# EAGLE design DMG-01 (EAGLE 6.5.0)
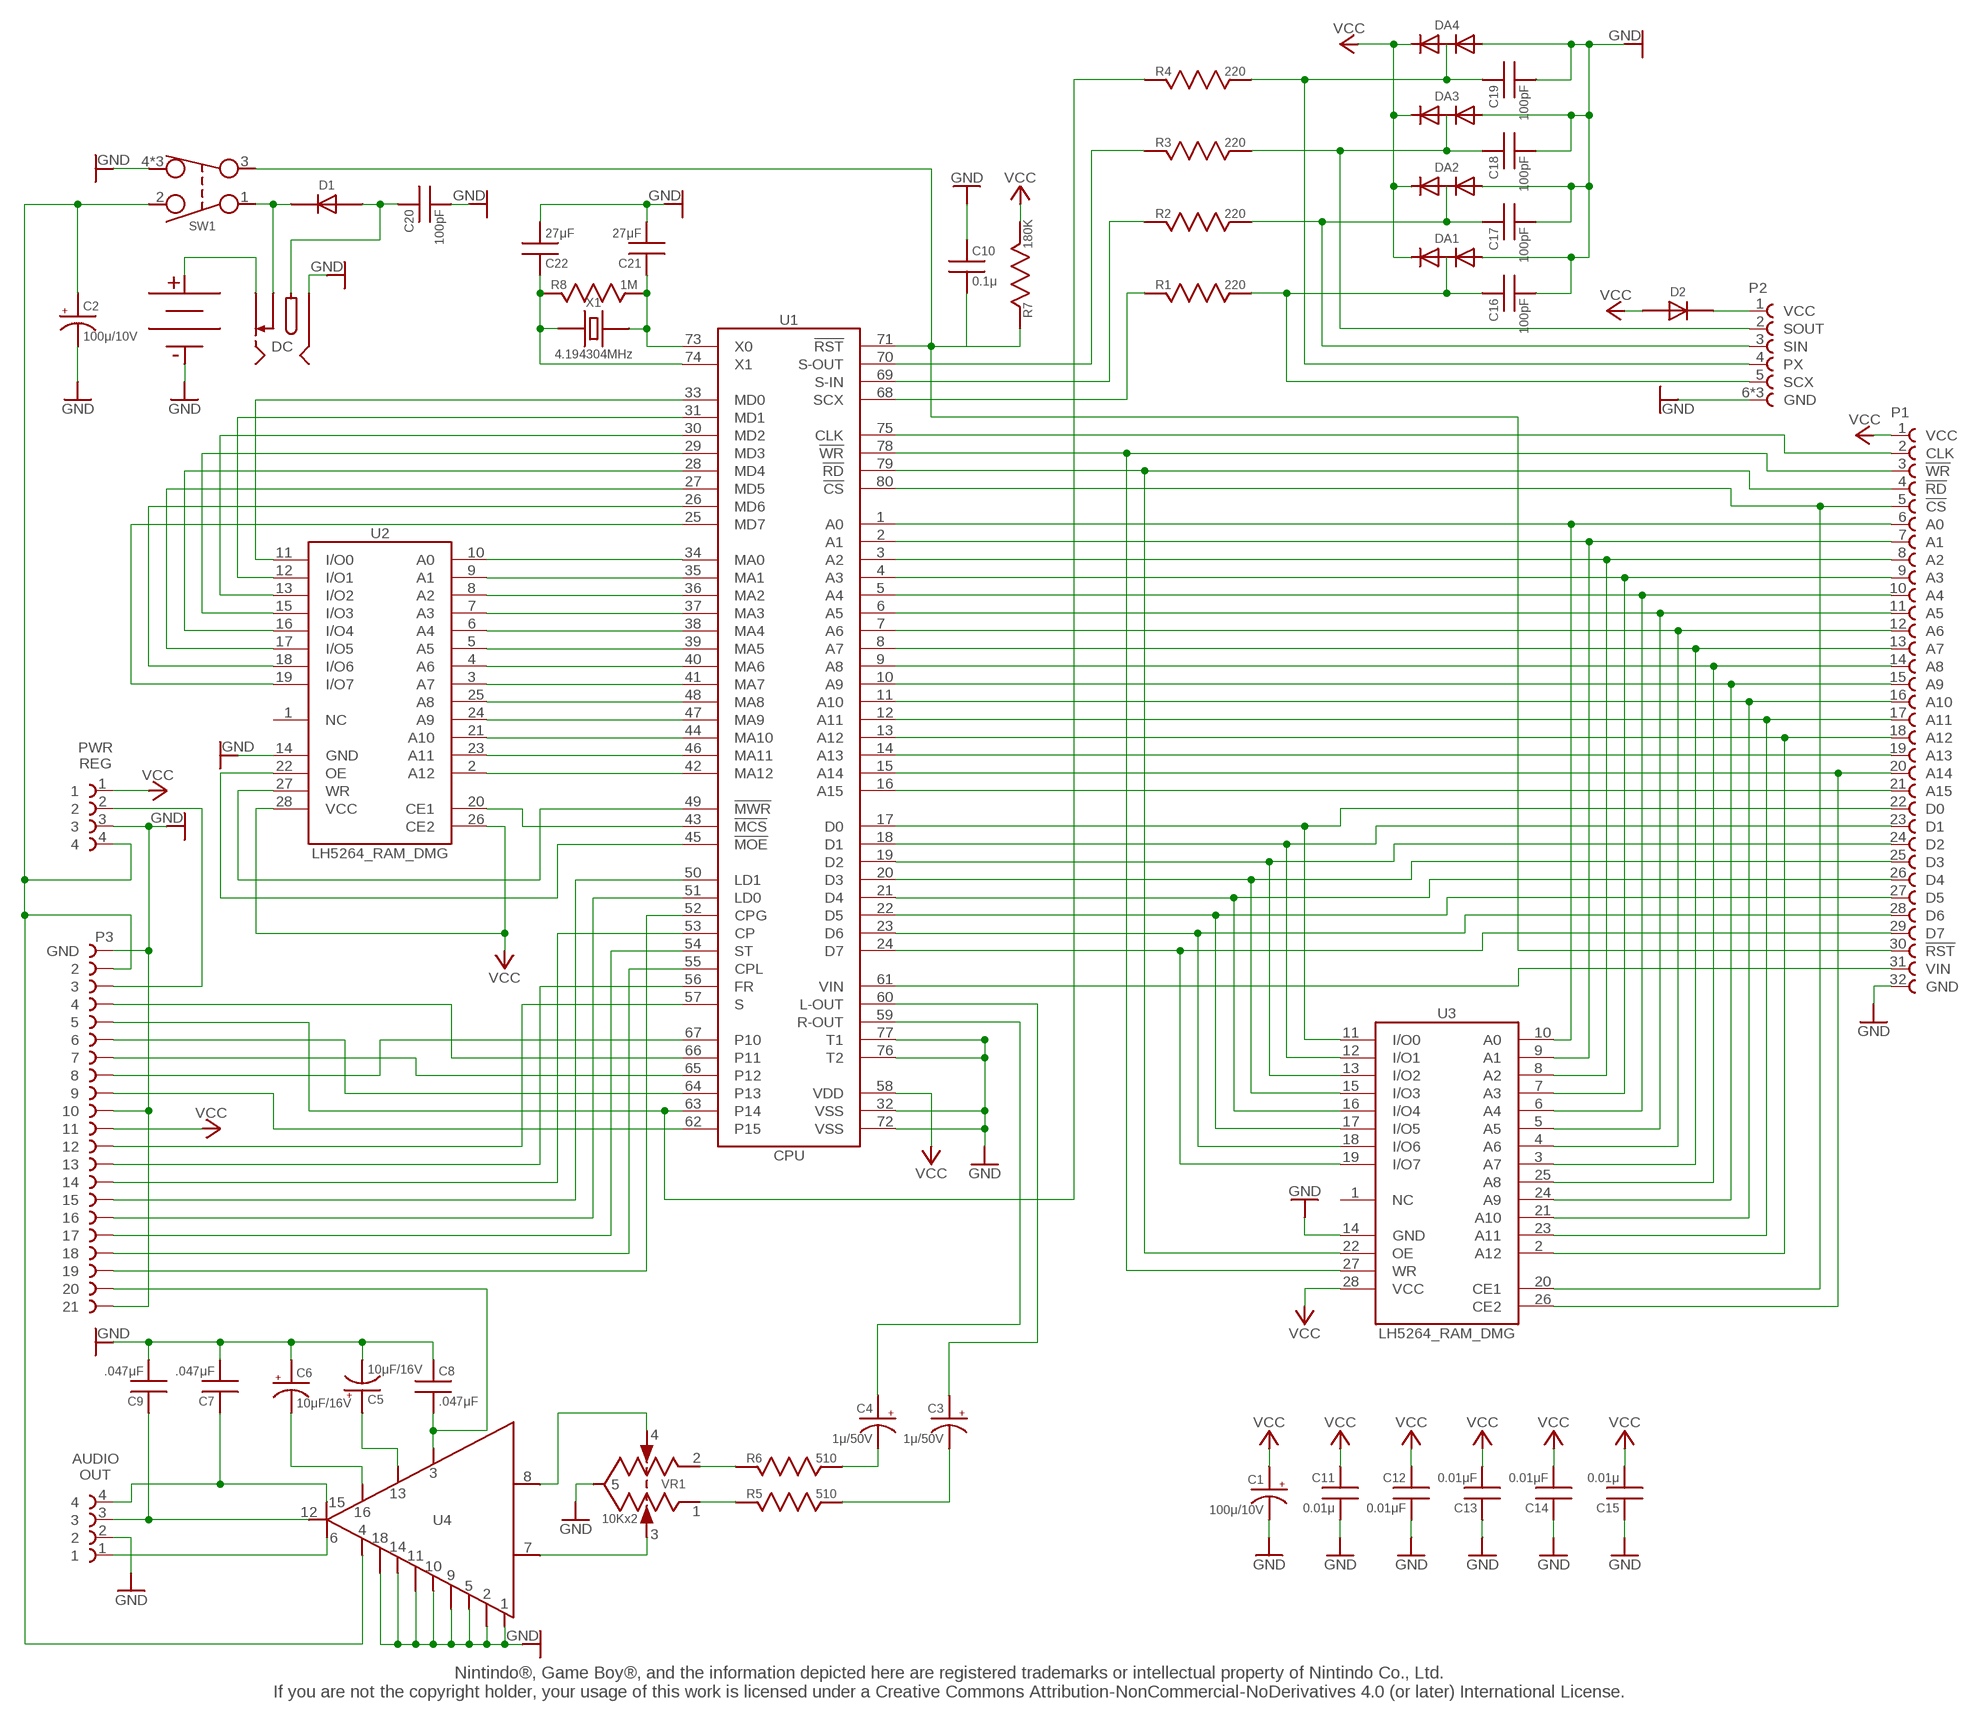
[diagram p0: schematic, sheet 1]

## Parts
C1  100μ/10V  CAPACITOR_ELECTROLYTIC_200MIL  [CAP-200E]
C2  100μ/10V  CAPACITOR_ELECTROLYTIC_200MIL  [CAP-200E]
C3  1μ/50V  CAPACITOR_ELECTROLYTIC_200MIL  [CAP-200E]
C4  1μ/50V  CAPACITOR_ELECTROLYTIC_200MIL  [CAP-200E]
C5  10μF/16V  CAPACITOR_ELECTROLYTIC_200MIL  [CAP-200E]
C6  10μF/16V  CAPACITOR_ELECTROLYTIC_200MIL  [CAP-200E]
C7  .047μF  CAPACITOR_200MIL  [CAP-200]
C8  .047μF  CAPACITOR_200MIL  [CAP-200]
C9  .047μF  CAPACITOR_200MIL  [CAP-200]
C10  0.1μ  CAPACITOR_200MIL  [CAP-200]
C11  0.01μ  CAPACITOR_200MIL  [CAP-200]
C12  0.01μF  CAPACITOR_200MIL  [CAP-200]
C13  0.01μF  CAPACITOR_200MIL  [CAP-200]
C14  0.01μF  CAPACITOR_200MIL  [CAP-200]
C15  0.01μ  CAPACITOR_200MIL  [CAP-200]
C16  100pF  CAPACITOR_100MIL  [CAP-100]
C17  100pF  CAPACITOR_100MIL  [CAP-100]
C18  100pF  CAPACITOR_100MIL  [CAP-100]
C19  100pF  CAPACITOR_100MIL  [CAP-100]
C20  100pF  CAPACITOR_100MIL  [CAP-100]
C21  27μF  CAPACITOR_100MIL  [CAP-100]
C22  27μF  CAPACITOR_100MIL  [CAP-100]
D1  DIODE_300MIL  [DIODE-300]
D2  DIODE_300MIL  [DIODE-300]
DA1  DIODE_ARRAY_DMG  [DMG_DIODE_ARRAY]
DA2  DIODE_ARRAY_DMG  [DMG_DIODE_ARRAY]
DA3  DIODE_ARRAY_DMG  [DMG_DIODE_ARRAY]
DA4  DIODE_ARRAY_DMG  [DMG_DIODE_ARRAY]
DC  PWR_JACK_DMG  [DMG_PWR_JACK]
P1  DMG_SOCKET  [DMG_SOCKET]
P2  DMG_LINK_PORT  [DMG_LINK_PORT]
P3  DMG_SOCKET_SCREEN  [DMG_SOCKET_SCREEN]
R1  220  RESISTOR600MIL  [RES-300]
R2  220  RESISTOR600MIL  [RES-300]
R3  220  RESISTOR600MIL  [RES-300]
R4  220  RESISTOR600MIL  [RES-300]
R5  510  RESISTOR600MIL  [RES-300]
R6  510  RESISTOR600MIL  [RES-300]
R7  180K  RESISTOR600MIL  [RES-300]
R8  1M  RESISTOR600MIL  [RES-300]
SW1  SWITCH_DMG  [DMG_SWITCH]
U1  CPU  LR35902_CPU_DMG  [LR35902_CPU_DMG]
U2  LH5264_RAM_DMG  [LH5264_RAM_DMG]
U3  LH5264_RAM_DMG  [LH5264_RAM_DMG]
U4  AMP_DMG  [AMP_DMG]
U$3  DMG_OUTBOARD  [DMG_OUTBOARD]
U$6  BAT+_DMG  [DMG_BAT+]
U$7  DMG_OUTBOARD  [DMG_OUTBOARD]
U$8  BAT-_DMG  [DMG_BAT-]
VR1  10Kx2  POT_DMG_DMG  [DMG_POT]
X1  4.194304MHz  CLOCK_DMG  [CLOCK_DMG]

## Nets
BAT: DC.4 U$6.POS(BAT+)
GND: C1.2(-) C2.2(-) C5.2(-) C6.1(+) C7.2 C8.1 C9.2 C10.1 C11.2 C12.2 C13.1 C14.1 C15.1 C16.2 C17.2 C18.2 C19.2 C20.2 C21.2 C22.2 DA1.1 DA2.1 DA3.1 DA4.1 DC.1 P1.32(GND) P2.6(GND) P2.MT1(GND) P2.MT2(GND) P3.1(GND) P3.10 P3.21 SW1.4 SW1.MT1 SW1.MT2 U1.32(VSS) U1.72(VSS) U1.76(T2) U1.77(T1) U2.14(GND) U3.14(GND) U4.1 U4.2 U4.5 U4.9 U4.10 U4.11 U4.14 U4.18 U$3.2 U$7.3 U$8.NEG(BAT-) VR1.5 VR1.MT1 VR1.MT2 ; supply symbol labelled GND_SIDE, GND_END
L-OUT: C3.1(+) U1.60(L-OUT)
L-STEP1: C3.2(-) R5.2
L-STEP2: R5.1 VR1.1
L-STEP3: U4.7 VR1.3
LEFT: C7.1 U4.15 U$3.4
N$1: P1.31(VIN) U1.61(VIN)
N$2: P3.3 U$7.2
N$3: D2.2 P2.1(VCC)
N$4: P1.29(D7) U1.24(D7) U3.19(I/O7)
N$5: P1.28(D6) U1.23(D6) U3.18(I/O6)
N$6: P1.27(D5) U1.22(D5) U3.17(I/O5)
N$7: P1.26(D4) U1.21(D4) U3.16(I/O4)
N$8: P1.25(D3) U1.20(D3) U3.15(I/O3)
N$9: P1.24(D2) U1.19(D2) U3.13(I/O2)
N$10: P1.23(D1) U1.18(D1) U3.12(I/O1)
N$11: P1.22(D0) U1.17(D0) U3.11(I/O0)
N$12: P1.21(A15) U1.16(A15)
N$13: P1.20(A14) U1.15(A14) U3.26(CE2)
N$14: P1.19(A13) U1.14(A13)
N$15: P1.18(A12) U1.13(A12) U3.2(A12)
N$16: P1.17(A11) U1.12(A11) U3.23(A11)
N$17: P1.16(A10) U1.11(A10) U3.21(A10)
N$18: P1.15(A9) U1.10(A9) U3.24(A9)
N$19: P1.14(A8) U1.9(A8) U3.25(A8)
N$20: P1.13(A7) U1.8(A7) U3.3(A7)
N$21: P1.12(A6) U1.7(A6) U3.4(A6)
N$22: P1.11(A5) U1.6(A5) U3.5(A5)
N$23: P1.10(A4) U1.5(A4) U3.6(A4)
N$24: P1.9(A3) U1.4(A3) U3.7(A3)
N$25: P1.8(A2) U1.3(A2) U3.8(A2)
N$26: P1.7(A1) U1.2(A1) U3.9(A1)
N$27: P1.6(A0) U1.1(A0) U3.10(A0)
N$28: P1.5(!CS) U1.80(!CS) U3.20(CE1)
N$29: P1.4(!RD) U1.79(!RD) U3.22(OE)
N$30: P1.2(CLK) U1.75(CLK)
N$31: U1.33(MD0) U2.11(I/O0)
N$32: U1.31(MD1) U2.12(I/O1)
N$33: U1.30(MD2) U2.13(I/O2)
N$34: U1.29(MD3) U2.15(I/O3)
N$35: U1.28(MD4) U2.16(I/O4)
N$36: U1.27(MD5) U2.17(I/O5)
N$37: U1.26(MD6) U2.18(I/O6)
N$38: U1.25(MD7) U2.19(I/O7)
N$39: U1.45(!MOE) U2.22(OE)
N$40: U1.49(!MWR) U2.27(WR)
N$41: U1.43(!MCS) U2.20(CE1)
N$42: U1.42(MA12) U2.2(A12)
N$43: U1.46(MA11) U2.23(A11)
N$44: U1.44(MA10) U2.21(A10)
N$45: U1.47(MA9) U2.24(A9)
N$46: U1.48(MA8) U2.25(A8)
N$47: U1.41(MA7) U2.3(A7)
N$48: U1.40(MA6) U2.4(A6)
N$49: U1.39(MA5) U2.5(A5)
N$50: U1.38(MA4) U2.6(A4)
N$51: U1.37(MA3) U2.7(A3)
N$52: U1.36(MA2) U2.8(A2)
N$53: U1.35(MA1) U2.9(A1)
N$54: U1.34(MA0) U2.10(A0)
N$55: C21.1 R8.2 U1.73(X0) X1.2
N$56: C22.1 R8.1 U1.74(X1) X1.1
N$57: P1.3(!WR) U1.78(!WR) U3.27(WR)
N$58: R3.1 U1.70(S-OUT)
N$59: R2.1 U1.69(S-IN)
N$60: P3.5 R4.1 U1.63(P14)
N$61: R1.1 U1.68(SCX)
N$62: C16.1 DA1.2 P2.5(SCX) R1.2
N$63: C17.1 DA2.2 P2.3(SIN) R2.2
N$64: C18.1 DA3.2 P2.2(SOUT) R3.2
N$65: C19.1 DA4.2 P2.4(PX) R4.2
N$77: U4.6 U$3.1
N$78: C6.2(-) U4.16
N$79: C8.2 P3.20 U4.3
N$80: P3.4 U1.66(P11)
N$81: P3.6 U1.64(P13)
N$82: P3.7 U1.65(P12)
N$83: P3.8 U1.67(P10)
N$84: P3.9 U1.62(P15)
N$85: P3.12 U1.57(S)
N$86: P3.13 U1.56(FR)
N$87: P3.14 U1.53(CP)
N$88: P3.15 U1.50(LD1)
N$89: P3.16 U1.51(LD0)
N$90: P3.17 U1.54(ST)
N$91: P3.18 U1.55(CPL)
N$92: P3.19 U1.52(CPG)
N$102: C5.1(+) U4.13
N$106: C20.1 D1.1 DC.2
PWR: C2.1(+) D1.2 DC.3 P3.2 SW1.1 SW1.2 U4.4 U$7.4
R-OUT: C4.1(+) U1.59(R-OUT)
R-STEP1: C4.2(-) R6.2
R-STEP2: R6.1 VR1.2
R-STEP3: U4.8 VR1.4
RIGHT: C9.1 U4.12 U$3.3
RST: C10.2 P1.30(!RST) R7.1 SW1.3 U1.71(!RST)
VCC: C1.1(+) C11.1 C12.1 C13.2 C14.2 C15.2 D2.1 DA1.3 DA2.3 DA3.3 DA4.3 P1.1(VCC) P3.11 R7.2 U1.58(VDD) U2.26(CE2) U2.28(VCC) U3.28(VCC) U$7.1 ; supply symbol labelled VCC_END
Unconnected: U2.1(NC) U3.1(NC)

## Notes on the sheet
- PWR
  REG
- AUDIO
  OUT
- Nintindo®, Game Boy®, and the information depicted here are registered trademarks or intellectual property of Nintindo Co., Ltd.
  If you are not the copyright holder, your usage of this work is licensed under a Creative Commons Attribution-NonCommercial-NoDerivatives 4.0 (or later) International License.

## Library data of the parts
C1-C6 = !custom:CAPACITOR_ELECTROLYTIC: DMG Electrolytic Capacitor
C7-C22 = !custom:CAPACITOR: Capacitor.
D1 D2 = !custom:DIODE: Diodes.
DA1-DA4 = !custom:DIODE_ARRAY_DMG: Used in DMG-01 for link-port sanitization.
DC = !custom:PWR_JACK_DMG: DC Power Jack used in DMG.
P1 = !custom:DMG_SOCKET: DMG Socket 32 Pin Cartridge Socket used in DMG-01
P2 = !custom:DMG_LINK_PORT: DMG Link port; used to communicate with other Gameboys.
P3 = !custom:DMG_SOCKET_SCREEN: DMG Flex Cable Connecter This part does not have any spec that can be found. Part was measured with a caliper with a resolution of .5mil. Pad spacing is at 50mil.
R1-R8 = !custom:RESISTOR: Resistor.
SW1 = !custom:SWITCH_DMG: Power switch used in DMG.
U1 = !custom:LR35902_CPU: Sharp LR35902 CPU Z80/8080 Hybrid used in the DMG-01 The origional spec cannot be found, so assumptions are made. This thin quad flat pack (TQFP) uses a common spacing of 0.8mm between the pins. When compaired to a scaled photo, the solder pads match very closely.
U2 U3 = !custom:LH5264_RAM: LH5264 RAM Memory used in DMG-01 Original spec sheet cannot be found. This part is based off a currently used SHARP 28SOP footprint (SOP025-P-0450). When compared to scaled photo of DMG pads, this footprint's center of tolerance matches perfectly. Pads extended to 2mm.
U4 = !custom:AMP_DMG: Gameboy Audio Amp. There is no information on this that can be found. All measurements were taken with a caliper with a resolution of 0.01mm/.5mil. Measurements were attempted in both mm and mil. The closest round number was chosen for every dimension, then re-measured for accuracy.
U$3 U$7 = !custom:DMG_OUTBOARD: Solder holes for connections to auxiliary boards.
U$6 = !custom:BAT+_DMG: Positive battery contact for DMG.
U$8 = !custom:BAT-_DMG: Negative battery contact for DMG.
VR1 = !custom:POT_DMG: Volume/Contrast Potentiomentor used on DMG-01. Based off a common thumb-wheel potentiometer that matches board.
X1 = !custom:CLOCK: Crystal Oscillator.

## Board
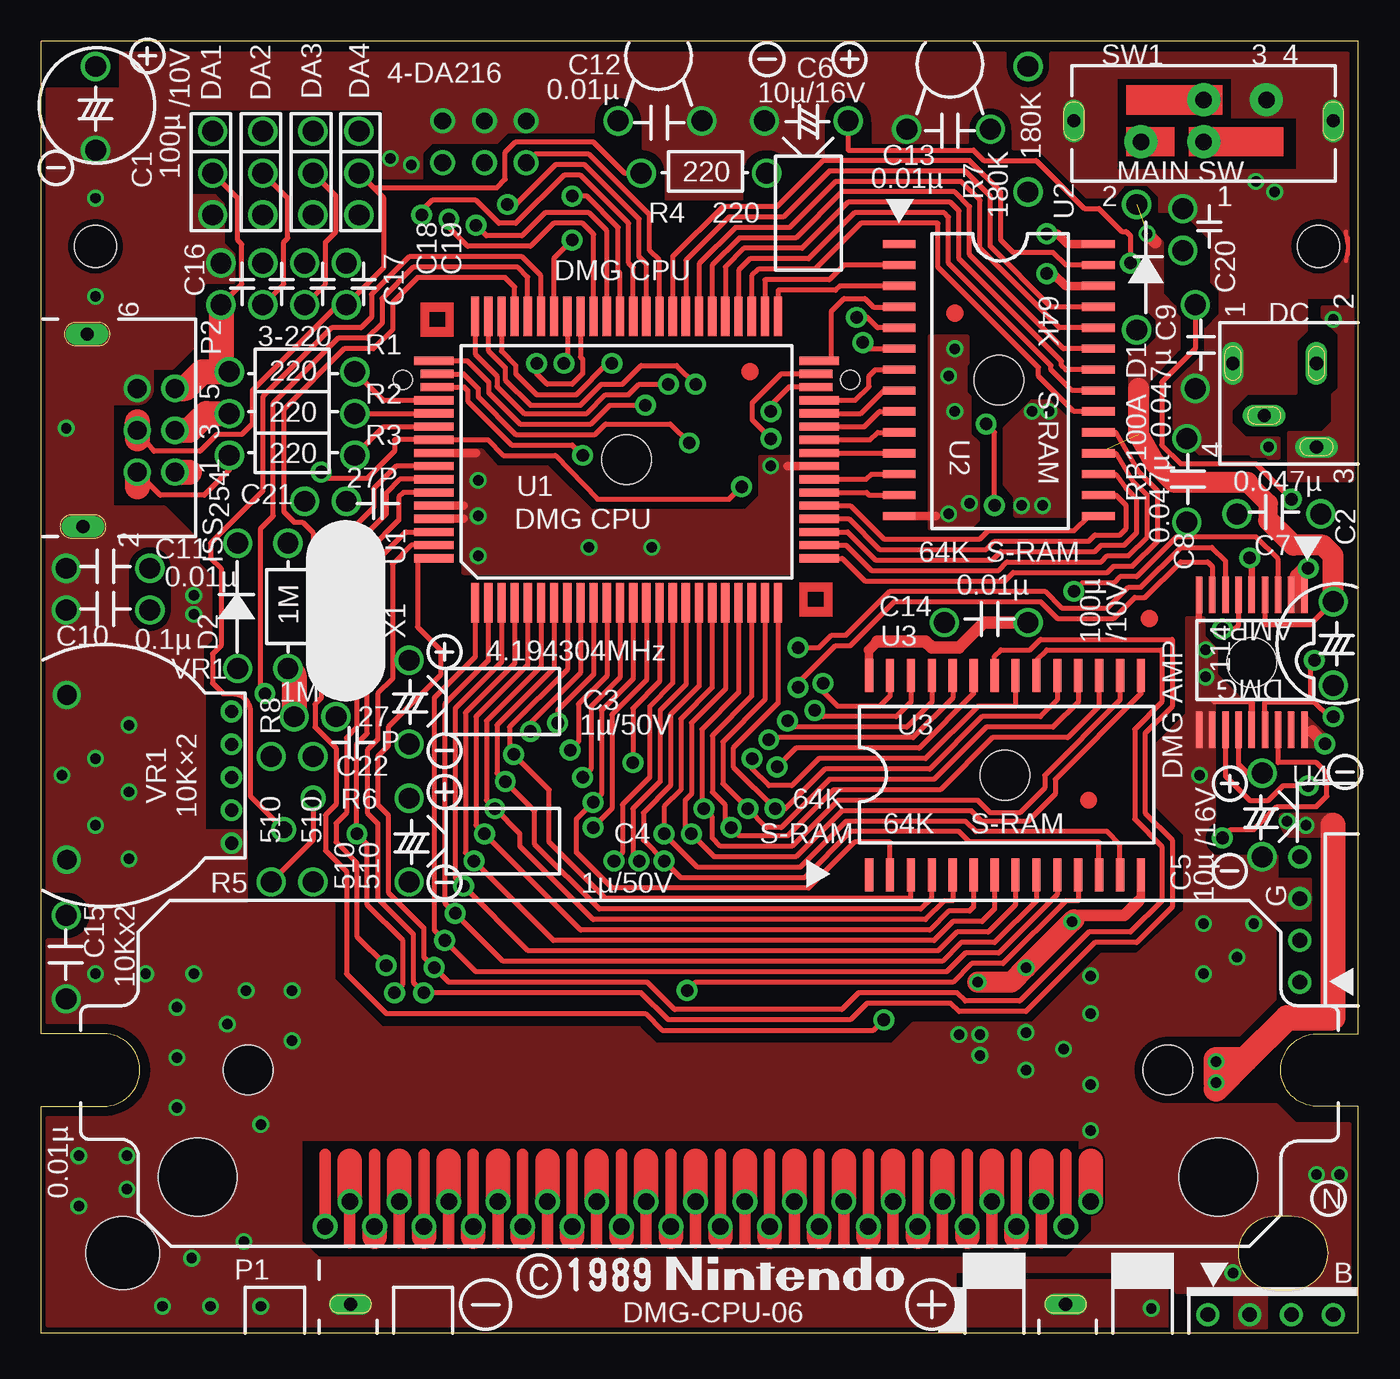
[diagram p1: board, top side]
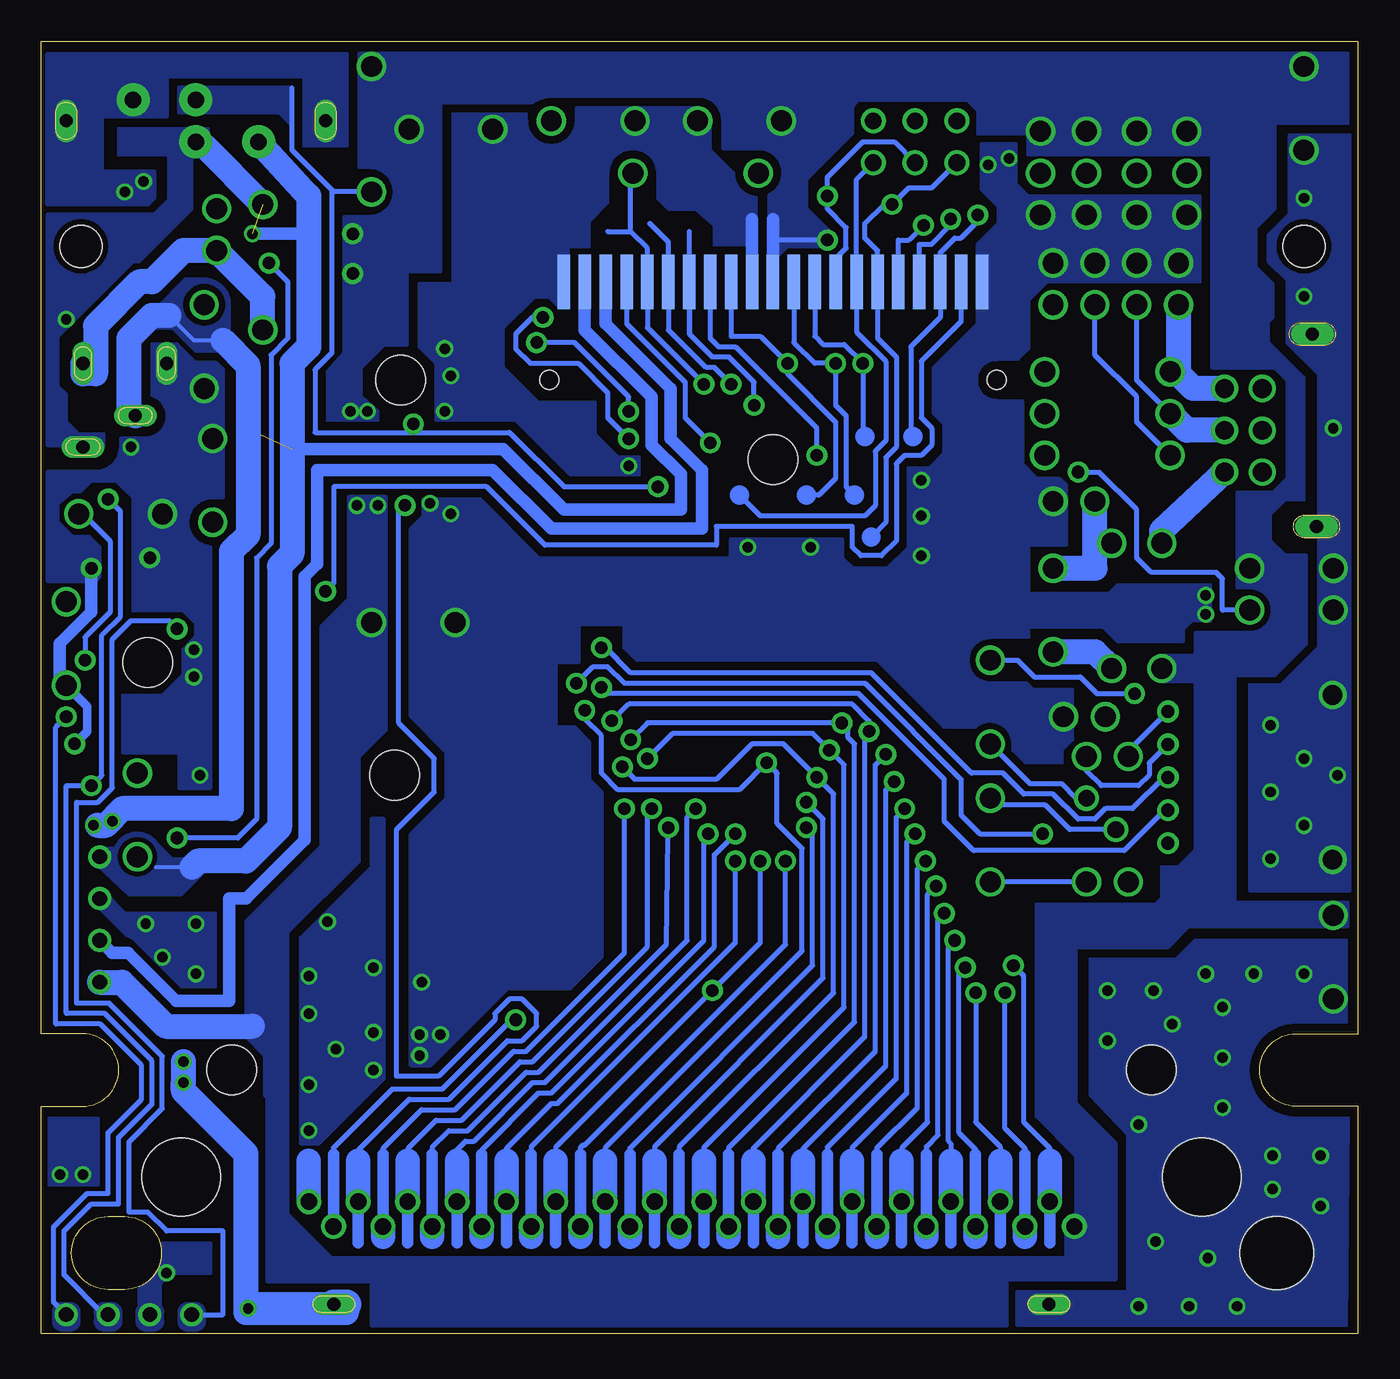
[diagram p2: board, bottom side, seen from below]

Size 80 x 78.5 mm. Coordinates in mm from the lower left corner, seen from the top.
Outline: 80,0 80,13.8 77.5,13.8 arc-180 77.5,18.2 80,18.2 80,78.5 0,78.5 0,18.2 3.8,18.2 arc-180 3.8,13.8 0,13.8 0,0 80,0
Copper layers (1*16): Top 0.035mm / dielectric 1.5mm / Bottom 0.035mm
Design rules "default *": minimum track width 10mil, minimum drill 24mil, track to track 5mil, track to pad 5mil, pad to pad 5mil, via to via 5mil, smd to smd 5mil, copper to edge 0mil, drill to drill 8mil, minimum pad ring 10mil, minimum via ring 1mil, stop-mask expansion 0mil, vias tented up to drill 0mil, thermal gap 0mil
Holes 2.54 mm at 3.3,66.04 77.6,66.04
Holes 4.45 mm at 4.95,4.89
Milling: 4 lines

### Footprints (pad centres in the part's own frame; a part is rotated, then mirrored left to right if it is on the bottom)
CAP-200E = drill 1.27: 1 -2.54,0; 2 2.54,0
CAP-200 = drill 1.27: 1 -2.54,0; 2 2.54,0
CAP-100 = drill 1.27: 1 -1.27,0; 2 1.27,0
DIODE-300 = drill 1.27: 1 3.81,0; 2 -3.81,0
DMG_DIODE_ARRAY = drill 1.27: 1 -2.54,0; 2 0,0; 3 2.54,0
DMG_PWR_JACK = drill 0.8 long: 1 -1.905,-2.54; 2 -1.905,2.54; 3 3.175,2.54; 4 1.27,-0.635
DMG_SOCKET = drill 1 pad 1.5: 1 -23.25,-9.5; 2 -21.75,-8; 3 -20.25,-9.5; 4 -18.75,-8; 5 -17.25,-9.5; 6 -15.75,-8; 7 -14.25,-9.5; 8 -12.75,-8; 9 -11.25,-9.5; 10 -9.75,-8; 11 -8.25,-9.5; 12 -6.75,-8; 13 -5.25,-9.5; 14 -3.75,-8; 15 -2.25,-9.5; 16 -0.75,-8; 17 0.75,-9.5; 18 2.25,-8; 19 3.75,-9.5; 20 5.25,-8; 21 6.75,-9.5; 22 8.25,-8; 23 9.75,-9.5; 24 11.25,-8; 25 12.75,-9.5; 26 14.25,-8; 27 15.75,-9.5; 28 17.25,-8; 29 18.75,-9.5; 30 20.25,-8; 31 21.75,-9.5; 32 23.25,-8 | hole 3: -27.925,0; 27.925,0 | hole 4.75: -31,-6.5; 31,-6.5
DMG_LINK_PORT = drill 1.143 pad 1.422: 1 7.366,-2.54; 2 5.08,-2.54; 3 7.366,0; 4 5.08,0; 5 7.366,2.54; 6 5.08,2.54 | drill 0.8 long: MT1 1.778,-5.842; MT2 2.032,5.842
DMG_SOCKET_SCREEN = smd 0.762 x 3.302: 1 -12.7,5.969; 2 -11.43,5.969; 3 -10.16,5.969; 4 -8.89,5.969; 5 -7.62,5.969; 6 -6.35,5.969; 7 -5.08,5.969; 8 -3.81,5.969; 9 -2.54,5.969; 10 -1.27,5.969; 11 0,5.969; 12 1.27,5.969; 13 2.54,5.969; 14 3.81,5.969; 15 5.08,5.969; 16 6.35,5.969; 17 7.62,5.969; 18 8.89,5.969; 19 10.16,5.969; 20 11.43,5.969; 21 12.7,5.969 | hole 1.143: -13.589,0; 13.589,0
RES-300 = drill 1.27: 1 -3.81,0; 2 3.81,0
DMG_SWITCH = drill 1 pad 2: 1 0,-1.27; 2 -3.81,-1.27; 3 0,1.27; 4 3.81,1.27 | drill 0.8 long: MT1 -7.874,0; MT2 7.874,0
LR35902_CPU_DMG = smd 0.5 x 2.4: 1 -9.2,-8.7; 2 -8.4,-8.7; 3 -7.6,-8.7; 4 -6.8,-8.7; 5 -6,-8.7; 6 -5.2,-8.7; 7 -4.4,-8.7; 8 -3.6,-8.7; 9 -2.8,-8.7; 10 -2,-8.7; 11 -1.2,-8.7; 12 -0.4,-8.7; 13 0.4,-8.7; 14 1.2,-8.7; 15 2,-8.7; 16 2.8,-8.7; 17 3.6,-8.7; 18 4.4,-8.7; 19 5.2,-8.7; 20 6,-8.7; 21 6.8,-8.7; 22 7.6,-8.7; 23 8.4,-8.7; 24 9.2,-8.7; 41 9.2,8.7; 42 8.4,8.7; 43 7.6,8.7; 44 6.8,8.7; 45 6,8.7; 46 5.2,8.7; 47 4.4,8.7; 48 3.6,8.7; 49 2.8,8.7; 50 2,8.7; 51 1.2,8.7; 52 0.4,8.7; 53 -0.4,8.7; 54 -1.2,8.7; 55 -2,8.7; 56 -2.8,8.7; 57 -3.6,8.7; 58 -4.4,8.7; 59 -5.2,8.7; 60 -6,8.7; 61 -6.8,8.7; 62 -7.6,8.7; 63 -8.4,8.7; 64 -9.2,8.7 | smd 2.4 x 0.5: 25 11.7,-6; 26 11.7,-5.2; 27 11.7,-4.4; 28 11.7,-3.6; 29 11.7,-2.8; 30 11.7,-2; 31 11.7,-1.2; 32 11.7,-0.4; 33 11.7,0.4; 34 11.7,1.2; 35 11.7,2; 36 11.7,2.8; 37 11.7,3.6; 40 11.7,6; 65 -11.7,6; 68 -11.7,3.6; 69 -11.7,2.8; 70 -11.7,2; 71 -11.7,1.2; 72 -11.7,0.4; 73 -11.7,-0.4; 74 -11.7,-1.2; 75 -11.7,-2; 76 -11.7,-2.8; 77 -11.7,-3.6; 78 -11.7,-4.4; 79 -11.7,-5.2; 80 -11.7,-6 | smd 2 x 0.5: 38 11.5,4.4; 39 11.5,5.2; 66 -11.5,5.2; 67 -11.5,4.4 | hole 3: 0,0
LH5264_RAM_DMG = smd 2 x 0.5: 1 -6.046,8.255; 2 -6.046,6.985; 3 -6.046,5.715; 4 -6.046,4.445; 5 -6.046,3.175; 6 -6.046,1.905; 7 -6.046,0.635; 8 -6.046,-0.635; 9 -6.046,-1.905; 10 -6.046,-3.175; 11 -6.046,-4.445; 12 -6.046,-5.715; 13 -6.046,-6.985; 14 -6.046,-8.255; 15 6.046,-8.255; 16 6.046,-6.985; 17 6.046,-5.715; 18 6.046,-4.445; 19 6.046,-3.175; 20 6.046,-1.905; 21 6.046,-0.635; 22 6.046,0.635; 23 6.046,1.905; 24 6.046,3.175; 25 6.046,4.445; 26 6.046,5.715; 27 6.046,6.985; 28 6.046,8.255 | hole 3: 0,0
AMP_DMG = smd 2.2 x 0.4: 1 -4.1,3.2; 2 -4.1,2.4; 3 -4.1,1.6; 4 -4.1,0.8; 5 -4.1,0; 6 -4.1,-0.8; 7 -4.1,-1.6; 8 -4.1,-2.4; 9 -4.1,-3.2; 10 4.1,-3.2; 11 4.1,-2.4; 12 4.1,-1.6; 13 4.1,-0.8; 14 4.1,0; 15 4.1,0.8; 16 4.1,1.6; 17 4.1,2.4; 18 4.1,3.2 | hole 3: 0,0
DMG_OUTBOARD = drill 0.889: 1 -3.81,0; 2 -1.27,0; 3 1.27,0; 4 3.81,0
DMG_BAT+ = drill 0.8 long: POS 0,0
DMG_BAT- = drill 0.8 long: NEG 0,0
DMG_POT = drill 0.8: 1 -4,7.5; 2 -2,7.5; 3 0,7.5; 4 2,7.5; 5 4,7.5 | drill 1.2: MT1 -5,-2.5; MT2 5,-2.5
CLOCK_DMG = drill 1.27: 1 -2.54,0; 2 2.54,0

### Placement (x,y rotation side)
C1  3.3,74.42 270 top
C2  78.49,41.91 270 top
C3  22.35,38.35 270 top
C4  22.35,29.97 270 top
C5  74.17,31.5 270 top
C6  46.48,73.66 0 top
C7  75.18,49.78 180 top
C8  69.6,51.82 270 top
C9  70.1,59.94 270 top
C10  4.06,43.94 0 top
C11  4.06,46.48 180 top
C12  37.59,73.66 0 top
C13  55.12,73.15 0 top
C14  57.4,43.18 0 top
C15  1.52,22.86 90 top
C16  10.92,63.75 90 top
C17  13.46,63.75 90 top
C18  16,63.75 90 top
C19  18.54,63.75 90 top
C20  69.34,67.06 90 top
C21  16.64,37.47 0 top
C22  17.27,50.55 0 top
D1  66.55,64.77 270 top
D2  11.94,44.2 270 top
DA1  10.41,70.48 90 top
DA2  13.46,70.48 90 top
DA3  16.51,70.48 90 top
DA4  19.3,70.48 90 top
DC  74.93,57.02 270 top
P1  40.5,16 0 top
P2  0.76,54.86 0 top
P3  35.56,57.91 0 bottom
R1  15.24,58.42 180 top
R2  15.24,55.88 180 top
R3  15.24,53.34 180 top
R4  40.26,70.48 180 top
R5  13.97,31.24 270 top
R6  16.51,31.24 270 top
R7  59.94,73.15 90 top
R8  14.99,44.2 270 top
SW1  70.61,73.66 0 top
U1  35.56,53.09 0 top
U2  58.17,57.91 0 top
U3  58.55,33.91 90 top
U4  73.53,40.77 270 top
U$3  74.68,1.14 0 top
U$6  62.23,1.78 0 top
U$7  76.45,25.15 90 top
U$8  18.8,1.78 0 top
VR1  4.06,33.78 270 top
X1  18.54,43.94 270 top

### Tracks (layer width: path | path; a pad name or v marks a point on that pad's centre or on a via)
BAT  (via drill 0.64 pad 1.02)
  Top 1.524: 73.15,16.64 71.37,14.86 v71.37,15.24 v71.37,16.51 71.37,16.64 73.15,16.64 | 73.15,16.64 75.69,19.18 78.49,19.18 78.49,30.86
  Bottom 0.254: 72.26,61.85 70.74,60.33 68.96,60.33
  Bottom 0.762: 76.58,30.86 v76.83,30.86
  Bottom 1.524: DC.4 74.68,56.13 74.68,60.45 73.28,61.85 72.26,61.85 | 68.96,60.33 67.44,58.8 67.44,48.51 68.45,47.5 68.45,31.88 75.06,31.88 76.07,30.86 76.58,30.86 | 61.47,1.78 61.47,1.27 67.56,1.27 67.56,1.78 | 67.56,1.78 U$6.POS | 67.56,1.78 67.56,10.92 71.37,14.73 v71.37,15.24 v71.37,16.51
  Bottom 1.778: U$6.POS 61.47,1.78
  other vias: 75.69,31.11 67.44,1.52
  pour Top: 56.26,3.3 56.26,0.38 68.45,0.38 68.45,3.3
  pour Bottom (rank 4): 70.61,59.69 68.58,59.69 68.58,62.48 arc-90 70.1,64.01 71.25,64.01 73.03,62.23 73.03,61.09 72.01,61.09
  pour Top (no thermals): 76.2,31.5 76.2,30.23 arc-3
  pour Top (no thermals): 78.49,31.24 75.44,31.24 75.82,30.48 78.49,30.48
  cutout Bottom (no thermals): 70.1,63.75 arc180 70.1,61.21 arc180
GND  (via drill 0.64 pad 1.02, 0.76 pad 1.27, 1.02 pad 1.52)
  Top 0.254: 79.38,66.55 79.38,66.17 | 79.38,66.17 79.38,65.91 | 79.38,65.91 79.38,65.53 | 79.38,66.17 79.25,66.93 | 79.38,65.91 79.25,65.15
  Top 0.305: U4.18 77.22,36.67 77.22,36.58
  Top 0.406: U4.9 70.33,43.33 70.36,43.31 | U4.5 73.53,46.99 v73.41,47.12 | U4.2 76.33,44.87 | 76.33,44.87 76.33,45.97 | 76.33,44.87 U4.1 | U4.14 73.53,38.3 73.41,38.43 71.25,38.43
  Top 0.508: U3.14 66.8,26.42 66.67,26.29 | U2.14 54.36,49.66 | U1.32 45.34,52.69 | U1.76 25.65,50.29 | U1.77 25.65,49.49 | U1.72 26.42,53.49
  Top 0.711: 66.67,26.29 65.79,25.4 62.99,25.4 62.74,25.15
  Top 0.762: 77.22,36.58 v77.98,35.81
  Top 1.016: v76.96,46.48 76.83,46.48 76.33,45.97
  Top 1.27: v56.9,21.34 58.93,21.34 v59.82,22.23 v62.61,25.02 62.74,25.15
  Bottom 0.508: C2.2 77.22,38.1 77.22,36.58 v77.98,35.81
  Bottom 0.762: P3.10 36.83,67.69 | C2.2 78.87,39.75 78.87,41.91 76.96,43.81 76.96,45.85
  other vias: 24.38,73.66 26.92,73.66 29.46,73.66 70.36,33.91 70.74,39.88 70.74,41.53 70.61,21.84 72.64,22.86 73.66,24.89 70.61,24.89 63.75,21.72 63.75,19.43 62.1,17.27 63.75,15.11 59.82,16 59.82,18.29 57.02,18.16 57.02,16.89 55.75,18.16 63.75,12.32 26.54,51.82 26.54,49.66 26.54,47.24 33.27,47.75 37.08,47.75 44.32,52.7 55.12,49.78 56.39,50.42 55.5,56.01 55.12,58.17 55.5,59.82 74.55,53.85 73.79,69.98 74.93,69.34 21.21,71.37 22.48,70.99 3.3,68.96 3.3,62.99 9.27,44.83 9.27,43.69 5.33,36.96 3.3,34.92 1.27,33.91 5.33,32.89 3.3,30.86 5.33,28.83 3.3,21.84 6.35,21.84 8.26,19.81 9.27,21.84 12.45,20.83 15.24,20.83 15.24,17.78 11.3,18.8 8.26,16.76 13.34,12.7 8.26,13.72 5.21,10.79 2.29,10.79 2.29,7.75 5.21,8.76 9.14,4.57 12.32,5.59 13.34,1.65 10.29,1.65 7.37,1.65 77.47,9.65 78.87,9.65 72.39,3.68 1.52,54.99
  pour Bottom (rank 3, no thermals): 47.88,20.95 51.69,20.95 56.39,16.26 57.53,16.26 57.53,30.35 55.37,32.51 55.37,35.31 57.53,37.47 57.53,48.9 56.77,49.66 56.77,50.67 53.34,50.67 49.78,47.12 38.1,47.12 38.1,48.26 31.37,48.26 31.37,47.12 30.73,46.48 28.57,46.48 27.3,47.75 27.3,52.58 26.04,52.58 25.15,53.47 25.15,55.24 25.78,55.88 25.78,58.67 23.11,61.34 23.11,66.17 21.84,67.44 21.84,68.45 22.86,69.47 22.86,72.26 20.83,72.26 20.83,69.85 20.07,69.09 9.65,69.09 9.65,63.88 18.92,63.88 20.07,62.74 20.07,59.82 20.7,59.18 21.97,59.18 arc-180 21.97,56.64 20.45,56.64 20.45,52.83 19.56,51.94 18.16,51.94 17.78,51.56 17.78,47.88 20.07,47.88 20.07,44.96 15.11,44.96 14.61,45.47 9.02,45.47 9.02,43.31 10.16,43.31 10.67,42.8 10.67,42.04 14.61,42.04 15.49,42.93 20.07,42.93 20.07,42.29 22.35,42.29 arc-180 22.35,39.5 20.19,39.5 19.81,39.12 17.4,39.12 17.4,36.07 18.03,35.43 18.03,34.67 20.19,34.67 20.95,35.43 20.95,35.81 arc-133 23.32,36.83 25.15,36.83 29.21,40.89 43.81,40.89 44.58,41.66 44.58,43.05 47.37,43.05 47.37,40.77 48.77,40.77 48.77,36.83 47.62,36.83 46.74,35.94 46.74,33.66 45.97,32.89 45.97,22.86
  pour Top (rank 4, no thermals): 0.38,0.51 55.5,0.51 55.5,3.81 68.96,3.81 68.96,2.54 72.52,2.54 72.52,0.38 74.42,0.38 74.42,2.54 79.5,2.54 79.5,12.7 76.2,12.7 75.06,13.84 68.45,13.84 arc-180 68.45,18.16 72.77,18.16 74.93,20.32 74.93,25.15 77.09,25.15 77.09,27.56 75.06,27.56 75.06,28.96 71.25,28.96 70.87,29.34 arc-100 71.25,31.11 71.25,38.35 73.03,38.35 71.37,40.01 71.37,41.53 70.61,42.29 70.61,43.43 69.6,43.43 69.6,37.59 67.69,35.69 67.69,32.13 69.47,30.35 69.47,25.65 66.55,22.99 64.39,22.99 60.2,18.8 52.96,18.8 51.69,17.53 37.34,17.53 36.32,18.54 20.7,18.54 17.78,21.46 17.78,26.04 12.45,26.04 12.45,30.48 9.91,30.48 9.91,38.99 9.78,39.12 9.78,41.66 10.29,42.16 10.29,45.97 9.53,46.74 9.53,48.13 7.49,50.16 4.32,50.16 4.32,56.52 5.84,56.52 arc90 6.73,57.4 6.73,58.67 8,58.67 9.27,59.94 9.27,63.12 10.03,63.88 11.68,63.88 11.68,65.53 11.05,66.17 11.05,68.58 10.54,69.09 8.89,69.09 8.89,74.42 20.83,74.42 20.83,70.23 23.11,70.23 23.11,71.75 23.75,72.39 27.69,72.39 28.32,73.03 33.53,73.03 33.53,73.66 arc-180 36.58,73.66 36.58,72.01 arc-90 37.97,70.48 37.97,68.96 42.55,68.96 42.55,70.61 arc-127 45.09,71.63 47.5,71.63 47.5,73.66 arc-180 50.55,73.66 50.55,72.39 56.26,72.39 56.26,73.15 arc-180 59.05,73.15 59.05,72.01 60.58,72.01 63.5,69.09 65.15,69.09 65.79,69.85 67.18,69.85 67.94,69.09 67.94,68.2 69.34,68.2 71.12,66.42 71.12,63.88 71.63,63.37 71.63,61.85 70.74,60.96 70.74,59.56 68.83,57.66 68.83,54.99 70.36,53.47 73.41,53.47 73.53,53.34 74.42,53.34 74.55,53.21 75.18,53.21 75.18,54.36 73.15,54.36 72.26,55.24 72.26,56.13 73.28,57.15 76.2,57.15 76.2,60.33 76.83,60.96 76.83,62.99 79.38,62.99 79.38,77.72 61.34,77.72 61.34,76.96 arc-180 58.55,76.96 58.55,77.72 4.83,77.72 4.83,75.56 0.38,75.56 0.38,26.92 1.52,26.92 arc-180 1.52,23.88 0.38,23.88 0.38,18.92 3.81,18.92 arc-180 3.81,13.08 0.38,13.08
  pour Bottom (no thermals): 56.01,55.5 51.18,55.5 47.88,52.2 43.69,52.2 43.69,53.21 44.96,53.21 46.35,54.61 46.35,56.52 49.78,56.52 51.94,58.67 51.94,61.09 50.04,62.99 49.15,62.99 48.51,62.36 48.01,62.36 48.01,66.04 46.74,66.04 46.74,67.56 45.59,68.71 45.59,70.48 arc180 42.55,70.48 42.55,68.96 41.91,68.33 40.26,68.33 39.12,67.31 39.12,66.17 36.58,66.17 36.58,68.96 arc85 37.97,70.48 39.37,71.88 39.37,73.41 arc-90 40.13,74.42 47.5,74.42 47.5,73.53 arc180 50.55,73.79 50.55,74.04 54.99,74.04 54.99,63.75 57.02,63.75 57.02,59.94 56.01,58.93
  pour Top: 53.98,60.58 56.26,60.58 56.26,58.93 56.13,58.8 56.13,57.15 56.39,56.9 56.39,54.61 56.9,54.1 56.9,49.4 56.39,48.9 53.98,48.9
  pour Bottom (no thermals): 69.72,33.15 69.72,47.75 arc175 69.6,50.8 68.96,50.8 68.96,58.55 69.34,58.93 70.61,58.93 71.75,60.07 73.28,60.07 73.28,57.02 arc160 73.66,54.36 75.18,54.36 75.18,53.85 arc90 76.71,52.32 79.63,52.32 79.63,45.72 76.71,45.72 76.45,45.97 76.45,47.75 77.09,48.39 78.11,48.39 78.99,49.28 78.99,50.42 78.11,51.18 77.6,51.18 76.96,51.82 75.44,51.82 74.42,50.8 74.42,43.94 71.37,43.94 70.61,43.18 70.61,42.29 71.37,41.53 71.37,40.01 72.64,38.73 75.06,38.73 75.06,35.31 71.63,35.31 71.63,33.15
  pour Bottom (no thermals): 69.47,25.53 69.47,21.08 71.48,21.08 74.4,24 74.8,24.2 76.76,26.16 arc184 76.13,26.72 74.93,25.53
  pour Bottom: 63.12,11.56 59.18,15.49 59.18,31.24 59.94,31.24 59.94,28.32 64.26,24 64.26,11.56
  pour Bottom (no thermals): 0.51,26.92 0.51,72.77 4.19,72.77 4.19,67.94 5.46,66.67 5.46,65.15 4.32,64.01 4.32,60.2 2.41,58.29 2.41,41.66 4.7,39.37 6.6,39.37 6.6,26.92
  pour Bottom (no thermals): 20.7,2.54 13.97,2.54 13.97,12.06 16.26,14.48 16.26,22.73 11.05,22.73 9.91,23.88 0.76,23.88 0.76,18.92 3.81,18.92 arc-180 3.81,13.08 0.64,13.08 0.76,0.51 20.7,0.51
  pour Top: 25.65,53.59 25.65,46.23 45.47,46.23 45.47,53.21 43.69,53.21 43.69,50.8 42.8,49.91 33.4,49.91 30.73,52.58 27.69,52.58 26.8,53.59
  pour Bottom (no thermals): 73.15,1.78 73.66,1.78 arc-90 74.17,1.27 74.17,0.76 arc-90 73.66,0.25 73.15,0.25 arc-90 72.64,0.76 72.64,1.27 arc-90
  pour Bottom (no thermals): 72.77,1.78 72.77,3.05 72.14,3.68 69.72,3.68 69.72,5.46 72.64,5.46 arc81 74.04,2.71 74.04,1.78
  pour Bottom (no thermals): 73.15,70.61 73.15,68.96 73.53,68.58 79.63,68.58 79.63,77.72 61.47,77.72 61.47,72.14 64.01,72.14 64.01,76.33 72.39,76.33 72.39,73.91 76.33,73.91 76.33,70.61
  pour Top (no thermals): 75.95,45.85 75.95,43.89 76.71,43.89 76.71,45.85
  pour Top (no thermals): 76.71,35.69 78.23,35.69 78.23,36.07 76.71,37.59
  cutout Top: 63.75,6.22 62.23,4.7 16.89,4.7 15.88,5.59 15.88,11.68 63,11.68 63,8 63.75,7.24
  pour Bottom (no thermals): 76.58,12.95 76.58,9.02 79.5,9.02 79.5,13.08 76.58,13.08
  cutout Top (no thermals): 72.26,73.79 76.2,73.79 76.2,70.74 65.41,70.74 65.41,76.2 72.26,76.2
  cutout Top (no thermals): 77.6,67.69 arc180 77.6,64.39 arc180
  cutout Bottom (no thermals): 3.3,67.69 arc180 3.3,64.39 arc180
  cutout Top (no thermals): 3.3,67.69 arc180 3.3,64.39 arc180
L-OUT  (via drill 0.76 pad 1.27)
  Top 0.305: U1.60 29.56,64.17 28.96,64.77 22.61,64.77 20.7,62.87 20.7,61.34 19.81,60.45 18.03,60.45 14.1,56.52 14.1,49.66 13.34,48.9 13.34,39.24 13.59,38.99 v13.59,38.86
  Bottom 0.305: C3.1 20.7,40.89 19.68,39.88 16.89,39.88 15.88,38.86 v13.59,38.86
L-STEP1  (via drill 1.02 pad 1.52)
  Top 0.305: v16.51,32.51 16.51,29.97 R5.2
  Bottom 0.305: C3.2 19.94,33.4 18.03,33.4 17.14,32.51 v16.51,32.51
L-STEP2
  Bottom 0.305: VR1.1 13.97,35.38 R5.1
L-STEP3  (via drill 0.76 pad 1.27)
  Top 0.305: v45.97,41.66 47.24,41.66 48.01,42.42 48.9,42.42 51.56,45.09 60.96,45.09 61.98,44.07 64.77,44.07 66.04,45.34 66.8,45.34 69.22,47.75 71.12,47.75 71.93,46.94 U4.7
  Bottom 0.305: VR1.3 11.81,33.78 13.72,31.88 15.37,31.88 16,31.24 17.02,31.24 18.54,32.77 20.32,32.77 21.59,34.04 23.5,34.04 29.59,40.13 44.2,40.13 45.72,41.66 v45.97,41.66
LEFT  (via drill 0.76 pad 1.27)
  Top 0.305: U4.15 74.33,38.35 77.09,38.35 | 77.09,38.35 77.34,38.35 78.23,37.47 v78.49,37.47 | v77.34,40.89 77.09,40.64 77.09,38.35
  Bottom 0.305: C7.1 77.47,49.78 75.82,48.13 75.82,43.81 77.34,42.29 v77.34,40.89 | U$3.4 79.25,1.91 79.25,6.48 77.22,8.51 75.95,8.51 75.95,12.19 73.91,14.22 73.91,16.27 76.44,18.8 79.12,18.8 79.12,36.83 v78.49,37.47
  pour Bottom (no thermals): 78.23,1.78 78.74,1.78 arc-90 79.25,1.27 79.25,0.76 arc-90 78.74,0.25 78.23,0.25 arc-90 77.72,0.76 77.72,1.27 arc-90
N$1  (via drill 0.76 pad 1.27)
  Top 0.305: U1.61 28.76,63.57 28.19,64.14 22.86,64.14 21.34,62.61 21.34,60.96 20.19,59.82 18.41,59.82 14.73,56.13 14.73,49.91 15.37,49.28 15.88,49.28 16.51,48.64 16.51,41.15 17.02,40.64 17.02,38.61 16.64,38.23 16.64,36.83 17.91,35.56 17.91,32.13 17.27,31.5 17.27,29.34 18.54,28.07 18.54,21.84 20.95,19.43 36.7,19.43 37.72,18.41 50.55,18.41 v51.18,19.05
  Bottom 0.305: v51.18,19.05 51.44,19.05 55.63,14.86 58.67,14.86 62.25,11.28 62.25,10.88
N$2
  Bottom 0.762: P3.3 45.72,61.34 41.78,57.4 41.78,54.36 39.88,52.45 39.88,48.9 49.02,48.9 52.58,52.45 63.25,52.45 63.25,46.74 64.01,45.97 64.01,29.97 67.56,26.42 68.58,26.42 68.58,20.19 71.81,20.19 74.73,23.11 75.69,23.11 U$7.2
N$3
  Top 1.524: P2.1 9.02,52.32
  Bottom 1.524: D2.2 11.94,48.77 P2.1
N$4  (via drill 0.76 pad 1.27)
  Top 0.305: U1.24 44.76,38.28 42.04,35.56 42.04,34.42 v44.58,31.88 45.21,31.88 47.62,34.29 53.98,34.29 57.15,37.47 60.71,37.47 61.72,38.48 U3.19
  Bottom 0.305: v44.58,31.88 44.58,23.11 50.55,17.14 51.31,17.14 54.86,13.59 56.9,13.59 59.25,11.23 59.25,10.88
N$5  (via drill 0.76 pad 1.27)
  Top 0.305: U1.23 43.96,38.5 41.4,35.94 41.4,33.4 v42.93,31.88 44.07,30.73 44.96,30.73 47.88,33.66 54.23,33.66 57.4,36.83 61.47,36.83 62.99,38.35 U3.18
  Bottom 0.305: v42.93,31.88 43.18,31.62 43.18,23.5 50.16,16.51 50.93,16.51 54.48,12.95 56.01,12.95 57.75,11.21 57.75,10.5
N$6  (via drill 0.76 pad 1.27)
  Top 0.305: U1.22 43.16,38.72 40.77,36.32 40.77,32.89 41.53,32.13 41.53,31.11 v41.91,30.73 42.42,30.23 45.34,30.23 48.13,33.02 54.61,33.02 57.78,36.2 62.36,36.2 64.26,38.1 U3.17
  Bottom 0.305: 41.92,30.23 42.04,23.62 49.78,15.88 50.55,15.88 54.1,12.32 55.24,12.32 56.25,11.31 56.25,10.88 | 41.92,30.23 v41.91,30.73 41.91,30.23 41.92,30.23
N$7  (via drill 0.76 pad 1.27)
  Top 0.305: U1.21 42.36,38.93 40.13,36.7 40.13,32 v40.26,31.88 40.77,31.37 40.77,30.1 41.27,29.59 45.59,29.59 48.39,32.38 56.9,32.38 57.66,31.62 59.44,31.62 60.96,33.15 60.96,33.91 65.53,38.48 U3.16
  Bottom 0.305: v40.26,31.88 40.77,31.37 40.77,23.88 49.4,15.24 50.16,15.24 53.72,11.68 54.23,11.68 54.75,11.16 54.75,10.5
N$8  (via drill 0.76 pad 1.27)
  Top 0.305: U1.20 41.56,39.15 39.5,37.08 39.5,32.77 39.12,32.38 39.12,30.73 v39.5,30.35 40.89,28.96 45.85,28.96 48.64,31.75 56.52,31.75 57.15,31.11 59.94,31.11 61.59,32.77 61.59,33.66 66.8,38.86 U3.15
  Bottom 0.305: v39.5,30.35 39.75,30.1 39.75,23.88 49.02,14.61 49.78,14.61 53.25,11.14 53.25,10.88
N$9  (via drill 0.76 pad 1.27)
  Top 0.305: U1.19 40.76,39.24 38.86,37.34 38.86,33.02 37.85,32 v37.85,30.35 39.88,28.32 46.1,28.32 48.9,31.11 56.13,31.11 56.77,30.48 64.77,30.48 65.53,29.72 U3.13
  Bottom 0.305: v37.85,30.35 39.12,29.08 39.12,23.5 48.64,13.97 49.02,13.97 51.75,11.24 51.75,10.5
N$10  (via drill 0.76 pad 1.27)
  Top 0.305: U1.18 39.96,39.33 38.23,37.59 38.23,33.27 36.58,31.62 36.58,29.97 v37.85,28.7 38.86,27.69 46.35,27.69 49.15,30.48 55.75,30.48 56.39,29.84 64.26,29.84 U3.12
  Bottom 0.305: v37.85,28.7 37.85,23.75 50.25,11.35 50.25,10.88
N$11  (via drill 0.76 pad 1.27)
  Top 0.305: U1.17 39.16,39.41 37.59,37.85 37.59,33.53 35.94,31.88 35.94,29.08 v36.32,28.7 | U3.11 62.99,26.29 62.23,26.29 58.42,22.48 56.52,22.48 55.37,21.34 39.75,21.34 v39.24,20.83
  Bottom 0.305: v36.32,28.7 36.32,23.75 v39.24,20.83 48.75,11.32 48.75,10.5
N$12  (via drill 0.76 pad 1.27)
  Top 0.305: U1.16 38.36,39.5 36.96,38.1 36.96,33.78 35.31,32.13 35.31,29.21 v34.8,28.7
  Bottom 0.305: v34.8,28.7 34.8,23.62 46.99,11.43 47.12,11.43 47.25,11.3 47.25,10.88
N$13  (via drill 0.76 pad 1.27)
  Top 0.305: U1.15 37.56,39.59 35.94,37.97 v35.94,34.67 | U3.26 52.83,38.35 51.94,37.47 47.5,37.47 v46.99,37.85
  Bottom 0.305: v46.99,37.85 46.99,37.34 45.97,36.32 45.97,34.04 44.96,33.02 37.59,33.02 v35.94,34.67 35.31,34.04 35.31,30.99 33.78,29.46 33.78,23.24 45.75,11.27 45.75,10.5
N$14  (via drill 0.76 pad 1.27)
  Top 0.305: U1.14 36.76,39.68 34.67,37.59 34.67,31.88 v33.53,30.73
  Bottom 0.305: v33.53,30.73 33.15,30.35 33.15,22.35 44.25,11.25 44.25,10.88
N$15  (via drill 0.76 pad 1.27)
  Top 0.305: U1.13 35.96,39.77 34.04,37.85 34.04,32.77 v33.53,32.26 32.51,31.24 32.51,29.21 34.67,27.05 46.61,27.05 49.4,29.84 51.56,29.84 U3.2
  Bottom 0.305: v33.53,32.26 32.51,31.24 32.51,21.59 42.75,11.35 42.75,10.5
N$16  (via drill 0.76 pad 1.27)
  Top 0.305: U1.12 35.16,39.86 33.4,38.1 33.4,34.29 v32.89,33.78 | U3.23 56.64,38.86 53.34,35.56 45.85,35.56 v44.7,34.42
  Bottom 0.305: v44.7,34.42 43.94,33.66 38.99,33.66 36.83,35.81 34.92,35.81 v32.89,33.78 31.88,32.77 31.88,20.7 41.25,11.33 41.25,10.88
N$17  (via drill 0.76 pad 1.27)
  Top 0.305: U1.11 34.36,39.95 32.64,38.23 32.64,35.94 v32.13,35.43 | U3.21 59.18,38.1 56.9,38.1 53.72,34.92 47.24,34.92 45.59,33.27 44.2,33.27 43.18,34.29 v43.18,34.92
  Bottom 0.305: v43.18,34.92 41.66,36.45 33.15,36.45 v32.13,35.43 31.24,34.54 31.24,19.81 39.75,11.3 39.75,10.5
N$18  (via drill 0.76 pad 1.27)
  Top 0.305: U1.10 33.56,40.04 31.37,37.85 v31.37,37.08 | U3.24 55.37,38.61 52.96,36.2 44.32,36.2 v44.2,36.07
  Bottom 0.305: v44.2,36.07 43.18,37.08 v31.37,37.08 30.99,36.7 30.99,36.2 30.61,35.81 30.61,18.92 38.25,11.28 38.25,10.88
N$19  (via drill 0.76 pad 1.27)
  Top 0.305: U1.9 32.76,40.13 29.72,37.08 v29.72,36.58 | U3.25 54.1,38.35 52.58,36.83 45.72,36.83 v45.34,37.21
  Bottom 0.305: v45.34,37.21 44.32,38.23 30.73,38.23 29.72,37.21 v29.72,36.58 29.97,36.32 29.97,18.03 36.75,11.26 36.75,10.5
N$20  (via drill 0.76 pad 1.27)
  Top 0.305: U1.8 31.96,40.34 28.45,36.83 28.45,35.43 v28.7,35.18 30.86,33.02 30.86,29.84 34.29,26.42 52.83,26.42 U3.3
  Bottom 0.305: v28.7,35.18 29.34,34.54 29.34,17.14 35.25,11.23 35.25,10.88
N$21  (via drill 0.76 pad 1.27)
  Top 0.305: U1.7 31.16,40.43 27.69,36.96 27.69,34.04 v28.19,33.53 29.97,31.75 29.97,29.72 33.91,25.78 53.42,25.78 54.1,26.47 U3.4
  Bottom 0.305: v28.19,33.53 28.7,33.02 28.7,16.26 33.75,11.21 33.75,10.5
N$22  (via drill 0.76 pad 1.27)
  Top 0.305: U1.6 30.36,40.52 27.05,37.21 27.05,32.38 v27.56,31.88 29.08,30.35 29.08,29.59 33.53,25.15 53.72,25.15 54.86,26.29 55.37,26.29 U3.5
  Bottom 0.305: v27.56,31.88 28.07,31.37 28.07,15.49 32.25,11.31 32.25,10.88
N$23  (via drill 0.76 pad 1.27)
  Top 0.305: U1.5 29.56,40.61 26.42,37.47 26.42,30.86 v26.92,30.35 32.77,24.51 53.98,24.51 55.12,25.65 56.39,25.65 56.64,25.91 U3.6
  Bottom 0.305: v26.92,30.35 27.43,29.84 27.43,14.61 30.75,11.29 30.75,10.5
N$24  (via drill 0.76 pad 1.27)
  Top 0.305: U1.4 28.76,40.7 25.78,37.72 25.78,29.21 v26.29,28.7 31.11,23.88 54.23,23.88 55.37,25.02 57.15,25.02 57.91,25.78 U3.7
  Bottom 0.305: v26.29,28.7 26.8,28.19 26.8,13.72 29.25,11.26 29.25,10.88
N$25  (via drill 0.76 pad 1.27)
  Top 0.305: U1.3 27.96,40.79 25.15,37.97 25.15,27.69 v25.65,27.18 29.59,23.24 54.48,23.24 55.63,24.38 57.53,24.38 59.18,26.04 U3.8
  Bottom 0.305: v25.65,27.18 26.16,26.67 26.16,12.83 27.75,11.24 27.75,10.5
N$26  (via drill 0.76 pad 1.27)
  Top 0.305: U1.2 27.16,40.88 24.51,38.23 24.51,26.16 v25.15,25.53 28.07,22.61 54.74,22.61 55.88,23.75 57.91,23.75 60.45,26.29 U3.9
  Bottom 0.305: v25.15,25.53 25.53,25.15 25.53,12.06 26.25,11.34 26.25,10.88
N$27  (via drill 0.76 pad 1.27)
  Top 0.305: U1.1 26.36,41.09 23.88,38.61 23.88,24.51 v24.51,23.88 26.42,21.97 54.99,21.97 56.13,23.11 58.17,23.11 61.72,26.67 U3.10
  Bottom 0.305: v24.51,23.88 24.89,23.5 24.89,11.68 24.75,11.54 24.75,10.5
N$28  (via drill 0.76 pad 1.27)
  Top 0.305: U1.80 22.86,47.09 22.86,42.93 24.26,41.53 24.26,40.01 21.08,36.83 21.08,35.69 20.45,35.05 20.45,32.13 21.08,31.5 21.08,26.8 23.24,24.64 23.24,22.86 v23.88,22.23 24.77,21.34 36.83,21.34 38.48,19.68 48.64,19.68 49.66,20.7 55.63,20.7 56.13,20.19 59.44,20.19 63.63,24.38 66.17,24.38 68.07,26.29 68.07,29.59 66.42,31.24 66.42,36.7 68.07,38.35 68.07,41.53 61.09,41.53 60.45,40.89 U3.20
  Bottom 0.305: v23.88,22.23 24.26,21.84 24.26,12.19 23.25,11.19 23.25,10.88
N$29  (via drill 0.76 pad 1.27)
  Top 0.305: U1.79 22.49,47.89 21.34,46.74 21.34,39.75 20.45,38.86 20.45,36.07 19.81,35.43 19.81,31.62 20.45,30.99 20.45,26.42 22.61,24.26 22.61,21.34 v23.24,20.7 36.45,20.7 38.1,19.05 49.15,19.05 50.16,20.07 55.24,20.07 55.75,19.56 59.82,19.56 64.01,23.75 66.55,23.75 68.71,25.91 68.71,29.97 67.06,31.62 67.06,36.45 68.71,38.1 68.71,42.16 60.71,42.16 60.07,41.53 58.29,41.53 57.91,41.15 U3.22
  Bottom 0.305: v23.24,20.7 23.24,12.83 21.75,11.34 21.75,10.5
N$30  (via drill 0.76 pad 1.27)
  Top 0.305: U1.75 22,51.09 21.72,50.8 21.72,49.4 19.94,47.62 19.94,40.64 19.18,39.88 19.18,36.83 18.54,36.2 18.54,31.62 17.91,30.99 17.91,29.84 19.18,28.57 19.18,24.13 v20.95,22.35
  Bottom 0.305: v20.95,22.35 20.32,21.72 20.32,12.83 18.75,11.26 18.75,10.5
N$31
  Top 0.305: U1.33 52.1,53.49 U2.11
N$32
  Top 0.305: U1.31 50.11,51.89 50.42,52.2 U2.12
N$33
  Top 0.305: U1.30 50.13,51.09 50.29,50.93 U2.13
N$34
  Top 0.305: U1.29 49.16,50.29 51.18,48.26 57.02,48.26 57.53,48.77 62.74,48.77 63.63,49.66 U2.15
N$35
  Top 0.305: U1.28 49.07,49.49 50.93,47.62 57.4,47.62 57.91,48.13 63.63,48.13 64.01,48.51 65.53,48.51 65.91,48.9 65.91,50.29 65.28,50.93 U2.16
N$36
  Top 0.305: U1.27 48.98,48.69 50.67,46.99 57.78,46.99 58.29,47.5 64.01,47.5 64.39,47.88 65.79,47.88 66.55,48.64 66.55,50.67 65.91,51.31 65.28,52.2 U2.17
N$37
  Top 0.305: U1.26 48.89,47.89 50.42,46.35 58.17,46.35 58.67,46.86 64.39,46.86 64.77,47.24 66.04,47.24 67.18,48.39 67.18,50.93 66.29,51.82 65.28,53.47 U2.18
N$38
  Top 0.305: U1.25 48.67,47.09 50.04,45.72 58.55,45.72 59.05,46.23 64.77,46.23 65.15,46.61 66.29,46.61 67.82,48.13 67.82,51.18 66.67,52.32 65.28,54.74 U2.19
N$39
  Top 0.305: U2.22 62.23,58.55 61.98,58.8 61.98,59.05 55.75,65.28 55.75,68.2 55.24,68.71 49.02,68.71 46.23,65.91 42.67,65.91 41.56,64.8 U1.45
N$40
  Top 0.305: U2.27 62.23,64.9 61.47,65.66 59.05,65.66 58.29,66.42 58.29,69.34 56.39,71.25 47.5,71.25 44.7,68.45 41.4,68.45 38.36,65.41 U1.49
N$41
  Top 0.305: U2.20 62.74,56.01 60.58,58.17 60.58,58.67 54.48,64.77 54.48,67.44 49.78,67.44 46.99,64.64 43.56,64.64 43.16,64.24 U1.43
N$42
  Top 0.305: U2.2 48.77,64.9 47.88,64.01 43.96,64.01 U1.42
N$43
  Top 0.305: U2.23 62.1,59.82 56.39,65.53 56.39,68.45 55.5,69.34 48.64,69.34 45.85,66.55 42.42,66.55 40.76,64.89 U1.46
N$44
  Top 0.305: U2.21 62.61,57.28 61.34,58.55 61.34,58.8 55.12,65.02 55.12,67.82 54.86,68.07 49.4,68.07 46.61,65.28 43.05,65.28 42.36,64.58 U1.44
N$45
  Top 0.305: U2.24 61.85,61.09 57.02,65.91 57.02,68.83 55.88,69.98 48.26,69.98 45.47,67.18 42.16,67.18 39.96,64.98 U1.47
N$46
  Top 0.305: U2.25 61.34,62.36 57.66,66.04 57.66,69.09 56.13,70.61 47.88,70.61 45.09,67.82 41.78,67.82 39.16,65.19 U1.48
N$47
  Top 0.305: U2.3 48.51,63.63 48.26,63.37 44.76,63.37 U1.41
N$48
  Top 0.305: U1.40 48.01,59.09 48.01,62.1 48.77,62.87 50.04,62.87 50.55,62.36 U2.4
N$49  (via drill 0.76 pad 1.27)
  Top 0.305: U1.39 44.95,58.29 43.18,56.52 43.18,55.5 v44.32,54.36 | U2.5 50.8,61.09 50.16,61.72 v49.53,61.72
  Bottom 0.305: v49.53,61.72 50.16,61.72 51.18,60.71 51.18,59.82 50.29,58.93 47.37,58.93 45.59,57.15 45.59,55.63 v44.32,54.36
N$50  (via drill 0.76 pad 1.27)
  Top 0.305: U1.38 45.42,57.49 44.32,56.39 v44.32,56.01 | v49.91,60.2 49.91,60.07 50.16,59.82 U2.6
  Bottom 0.305: v44.32,56.01 44.32,56.9 47.62,60.2 v49.91,60.2
N$51
  Top 0.305: U1.37 49.45,56.69 50.29,57.53 50.29,58.17 50.67,58.55 U2.7
N$52
  Top 0.305: U1.36 49.79,55.89 51.18,57.28 U2.8
N$53
  Top 0.305: U1.35 50.01,55.09 50.93,56.01 U2.9
N$54
  Top 0.305: U1.34 50.35,54.29 50.8,54.74 U2.10
N$55
  Top 0.305: U1.73 21.57,52.69 20.19,51.31 20.19,50.16 17.14,47.12 17.14,42.67 X1.2
  Top 1.524: R8.2 15.37,40.01 C21.1
  Bottom 1.524: R8.2 16,41.4 X1.2
N$56
  Top 0.305: U1.74 21.79,51.89 20.95,51.05 20.95,49.78 18.54,47.37 X1.1
  Bottom 1.524: X1.1 16,46.48 16,48.01 | 16,48.01 C22.1 | R8.1 16,48.01
N$57  (via drill 0.76 pad 1.27)
  Top 0.305: U3.27 51.56,38.73 50.93,38.1 48.39,38.1 47.5,38.99 v47.5,39.5 | U1.78 22.14,48.69 20.57,47.12 20.57,40.13 19.81,39.37 19.81,36.45 19.18,35.81 v19.18,30.35 19.81,29.72 19.81,26.04 21.97,23.88 21.97,21.21 v21.46,20.7
  Bottom 0.305: v21.46,20.7 21.46,12.45 20.25,11.23 20.25,10.88 | v47.5,39.5 46.48,40.51 45.59,40.51 44.58,39.5 29.97,39.5 24.13,33.66 24.13,31.5 22.99,30.35 v19.18,30.35
N$58
  Top 0.305: R3.1 20.8,55.09 U1.70
N$59
  Top 0.305: R2.1 U1.69
N$60  (via drill 0.76 pad 1.27)
  Top 0.305: U1.63 27.16,59.71 28.19,58.67 28.19,57.91 29.72,56.39 32.77,56.39 34.04,57.66 35.31,57.66 36.45,58.8 38.61,58.8 v39.75,57.66
  Bottom 0.305: 44.2,66.93 43.18,65.91 P3.5 43.18,61.09 v39.75,57.66 | 45.59,66.93 44.2,66.93 | 44.2,66.93 44.2,70.36 R4.1
N$61
  Top 0.305: R1.1 20.78,56.69 U1.68
N$62
  Top 0.305: C16.1 12.19,63.75 12.19,66.17 11.94,66.42 11.94,68.96 DA1.2
  Top 1.524: P2.5 8.76,57.4 9.78,58.42 10.92,58.42 | 10.92,58.42 R1.2 | C16.1 10.92,58.42
  Bottom 1.524: P2.5 10.03,57.4 10.92,58.29 10.92,58.42 | C16.1 10.92,58.42 | R1.2 10.92,58.42
N$63
  Top 0.305: C17.1 14.73,63.75 14.73,66.29 14.99,66.55 14.99,68.96 DA2.2
  Top 1.524: P2.3 9.02,54.86 10.03,55.88 R2.2
  Bottom 0.305: R2.2 13.46,57.91 C17.1
  Bottom 1.524: P2.3 10.41,54.86 R2.2
N$64
  Top 0.305: C18.1 17.27,63.75 17.27,66.29 17.91,66.93 17.91,69.09 DA3.2 | R3.2 11.43,52.45 9.91,50.93 7.24,50.93 P2.2
  Top 1.524: P2.2 5.84,51.44
  Bottom 0.305: R3.2 13.46,55.37 13.46,56.9 16,59.44 C18.1
N$65
  Top 0.305: DA4.2 20.19,69.6 | 20.19,69.6 27.69,69.6 28.19,70.1 28.19,71.75 28.83,72.39 33.53,72.39 35.43,70.48 R4.2 | 20.19,69.6 20.83,68.96 20.83,64.77 C19.1 18.03,62.48 12.83,57.28 12.83,55.24 12.19,54.61 10.67,54.61 9.65,53.59 6.86,53.59 P2.4
  Top 1.524: 5.84,54.36 P2.4 5.84,55.37
N$66  (via drill 1.02 pad 1.52)
  other vias: 26.92,71.12
N$67
  cutout Top (no thermals): 5.33,46.48 5.33,43.94 arc180 7.87,43.94 7.87,46.48 arc180
N$68  (via drill 1.02 pad 1.52)
  other vias: 24.38,71.12
N$69
  cutout Top (no thermals): 74.93,7.11 75.95,7.11 arc-180 75.95,2.67 74.93,2.67 arc-180
N$77  (via drill 0.76 pad 1.27)
  Top 0.305: U4.6 72.73,43.02 72.52,42.8 v71.75,42.8
  Bottom 0.305: U$3.1 68.96,1.14 68.96,6.22 72.39,6.22 73.53,7.37 74.68,7.37 74.68,11.63 72.64,13.66 72.64,16.84 75.87,20.07 77.85,20.07 77.85,32.26 76.58,32.26 75.69,33.15 75.69,42.16 74.55,43.31 72.26,43.31 v71.75,42.8
  pour Bottom (no thermals): 70.61,1.78 71.12,1.78 arc-90 71.63,1.27 71.63,0.76 arc-90 71.12,0.25 70.61,0.25 arc-90 70.1,0.76 70.1,1.27 arc-90
N$78  (via drill 0.76 pad 1.27)
  Top 0.305: C6.2 49.02,71.88 56.64,71.88 57.28,71.25 60.45,71.25 63.37,68.33 64.26,68.33 65.66,66.93 65.91,66.93 66.17,66.67 v66.17,65.02 | v71.75,30.1 72.26,30.61 73.66,30.61 75.06,32 77.47,32 78.11,32.64 78.11,34.04 77.47,34.67 75.13,34.67 U4.16
  Bottom 0.305: v66.17,65.02 65.02,63.88 65.02,60.45 66.04,59.44 66.04,48.01 66.93,47.12 66.93,31.24 68.07,30.1 v71.75,30.1
N$79  (via drill 0.76 pad 1.27)
  Top 0.305: U4.3 75.13,47.04 73.79,48.39 69.6,48.39 | 69.6,48.39 68.96,48.39 66.55,45.97 65.53,45.97 65.15,45.59 63.25,45.59 v62.74,45.09 | C8.2 69.6,48.39
  Bottom 0.305: P3.20 24.13,61.47 26.54,59.05 26.54,55.63 25.91,54.99 25.91,53.98 26.54,53.34 27.56,53.34 28.07,52.83 28.07,48.13 28.96,47.24 30.23,47.24 30.73,47.75 30.73,49.02 38.99,49.02 38.99,47.88 49.4,47.88 52.96,51.44 62.23,51.44 62.23,45.59 v62.74,45.09
N$80  (via drill 0.76 pad 1.27)
  Top 0.305: U1.66 25.66,58.29 26.54,57.4 26.54,56.9 28.83,54.61 33.66,54.61 34.29,55.24 38.23,55.24 v39.37,54.1
  Bottom 0.305: P3.4 44.45,61.34 40.89,57.78 40.89,55.63 v39.37,54.1
N$81  (via drill 0.76 pad 1.27)
  Top 0.305: U1.64 26.36,59.49 27.69,58.17 27.69,57.53 29.34,55.88 33.15,55.88 34.29,57.02 35.69,57.02 36.32,57.66 v38.1,57.66
  Bottom 0.305: 43.05,67.44 41.91,66.29 P3.6 41.91,60.96 39.62,58.67 39.12,58.67 v38.1,57.66
N$82  (via drill 0.76 pad 1.27)
  Top 0.305: U1.65 25.88,59.09 27.18,57.78 27.18,57.15 29.08,55.24 33.4,55.24 34.54,56.39 v36.7,56.39
  Bottom 0.305: P3.7 40.64,60.71 | 40.64,60.71 39.24,59.31 38.23,59.31 36.7,57.78 v36.7,56.39 | 40.64,60.71 | 40.64,60.71 40.64,66.93
N$83  (via drill 0.76 pad 1.27)
  Top 0.305: U1.67 25.7,57.49 25.91,57.28 25.91,56.64 28.57,53.98 32.26,53.98 v32.89,53.34
  Bottom 0.305: P3.8 39.37,60.45 38.86,59.94 37.85,59.94 32.89,54.99 v32.89,53.34
N$84  (via drill 0.76 pad 1.27)
  Top 0.305: U1.62 27.96,59.67 28.83,58.8 28.83,58.29 30.1,57.02 32.51,57.02 34.42,58.93 v34.67,58.93
  Bottom 0.305: P3.9 38.1,60.58 36.32,60.58 v34.67,58.93 34.67,58.29 31.75,55.37 31.75,51.94 32.77,50.93 33.53,50.93
N$85  (via drill 0.76 pad 1.27)
  Top 0.305: U1.57 31.96,59.14 v31.75,58.93
  Bottom 0.305: P3.12 34.29,60.2 33.02,58.93 v31.75,58.93 31.75,56.39 31.11,55.75 31.11,51.44 30.61,50.93
N$86  (via drill 0.76 pad 1.27)
  Top 0.305: U1.56 32.76,59.31 32.89,59.18 32.89,58.29 32.26,57.66 30.73,57.66 30.1,58.29 v30.1,58.93
  Bottom 0.305: P3.13 33.02,60.58 32.51,60.07 31.24,60.07 v30.1,58.93 30.1,54.48
N$87  (via drill 0.76 pad 1.27)
  Top 0.305: U1.53 35.16,64.41 35.05,64.52 35.05,67.18 33.15,69.09 v32.26,69.09
  Bottom 0.305: P3.14 31.75,65.28 31.11,65.91 31.11,67.18 32.26,68.33 v32.26,69.09 32.26,70.23 30.1,72.39 28.19,72.39 26.92,71.12
N$88  (via drill 1.02 pad 1.52)
  Top 0.305: U1.50 37.56,65.18 36.96,65.79 36.96,67.94 33.27,71.63 29.97,71.63 v29.46,71.12
  Bottom 0.305: v29.46,71.12 30.48,70.1 P3.15 30.48,60.83 28.7,59.05 28.7,54.23 29.34,53.59 29.34,50.29 29.97,49.66 36.32,49.66 37.47,50.8
N$89  (via drill 0.76 pad 1.27)
  Top 0.305: U1.51 36.76,64.97 36.32,65.41 36.32,67.69 33.02,70.99 31.24,70.99 28.83,68.58 v28.32,68.58
  Bottom 0.305: 24.38,71.12 25.91,69.6 27.3,69.6 v28.32,68.58 28.83,68.58 29.97,67.44 29.97,66.55 29.21,65.79 P3.16 29.21,60.45 28.07,59.31 28.07,53.85 28.7,53.21 28.7,49.28 29.59,48.39
N$90  (via drill 0.76 pad 1.27)
  Top 0.305: U1.54 34.36,66.99 33.27,68.07 30.61,68.07 29.21,66.67 27.05,66.67 v26.42,67.31
  Bottom 0.305: P3.17 27.94,66.42 27.3,66.42 v26.42,67.31
N$91  (via drill 0.76 pad 1.27)
  Top 0.305: U1.55 33.56,66.77 32.89,67.44 31.11,67.44 29.72,66.04 25.91,66.04 24.77,67.18 v24.77,67.69
  Bottom 0.305: P3.18 26.67,66.17 25.91,66.17 24.77,67.31 v24.77,67.69
N$92  (via drill 0.76 pad 1.27)
  Top 0.305: U1.52 35.96,64.75 35.69,65.02 35.69,67.44 32.77,70.36 31.75,70.36 28.83,67.44 27.81,67.44 26.42,68.83 23.75,68.83 23.11,68.2 v23.11,67.94
  Bottom 0.305: 26.92,54.36 27.18,54.61 27.18,59.94 25.4,61.72 P3.19 25.4,65.66 24.51,66.55 24.13,66.55 23.11,67.56 v23.11,67.94
N$102
  Top 0.305: U4.13 72.73,34.58 73.28,34.04 C5.1
N$106
  Bottom 1.524: D1.1 66.55,62.99 C20.1 71.37,65.79 73.28,63.88 74.04,63.88 76.71,61.21 76.71,58.29 77.47,58.29 DC.2
PWR  (via drill 0.64 pad 1.02)  (2 unrouted)
  Top 0.305: U4.4 74.33,43.05 77.09,43.05 C2.1
  Top 0.762: v67.18,66.8 67.69,66.29
  Top 1.143: 74.55,49.4 74.55,50.42 73.28,51.69
  Top 1.27: C2.1 78.49,47.24 77.85,47.88 76.07,47.88 74.55,49.4 | 73.28,51.69 68.83,51.69 67.69,52.83 66.67,54.61 66.67,57.4
  Bottom 0.254: 70.87,28.32 73.03,28.32
  Bottom 0.762: P3.2 46.99,60.96 42.93,56.9 42.93,53.98 41.15,52.2 41.15,50.04 48.26,50.04 51.94,53.72 64.77,53.72 | 63.75,69.09 63.75,66.8 v67.18,66.8
  Bottom 1.524: SW1.2 63.75,69.09 63.75,59.94 64.77,58.93 64.77,47.37 65.53,46.61 65.53,30.73 67.56,28.7 70.48,28.7 70.87,28.32 | D1.2 70.1,72.14 SW1.1
  other vias: 78.49,61.59
  pour Top (no thermals): 68.07,63.12 68.83,62.36 68.83,61.98 69.09,61.72 69.09,59.82 67.18,57.78 67.18,56.9 66.17,56.9 66.17,59.56 66.93,59.56 67.82,60.45 67.82,61.59 67.18,62.23 67.18,66.29 66.93,66.55 arc-203 67.44,66.93 68.07,66.29
  pour Bottom (no thermals): 76.58,29.46 75.44,29.46 73.28,30.02 72.09,28.83 71.12,28.83 70.1,28.07 71.5,26.67 74.68,26.67 76.58,28.45 arc147
  pour Bottom (no thermals): 79.63,53.98 76.2,53.98 76.2,54.61 77.72,54.61 78.49,55.37 78.49,57.02 78.99,57.53 78.99,60.58 74.42,65.15 74.04,65.15 70.87,68.33 70.87,71.5 69.85,71.5 69.85,73.15 75.31,73.15 75.31,71.63 72.26,71.63 72.26,68.83 73.15,67.94 79.63,67.94
  pour Top: 77.85,62.36 79.63,62.36 79.63,51.82 75.82,51.82 75.82,54.74 77.85,54.74 78.49,55.37 78.49,57.02 78.87,57.4 78.87,60.71 77.85,61.72
  cutout Bottom: 74.17,30.15 arc180 74.17,27.76 arc180
  pour Bottom (no thermals): 74.17,30.48 arc180 74.17,27.43 arc180
  pour Top (no thermals): 66.04,73.15 66.04,71.63 68.71,71.63 68.71,73.15
  pour Top (no thermals): 69.85,73.15 75.31,73.15 75.31,71.63 69.85,71.63
  cutout Bottom (no thermals): 77.6,67.69 arc180 77.6,64.39 arc180
R-OUT  (via drill 1.02 pad 1.52)
  Top 0.305: U1.59 30.36,64.25 29.21,65.41 22.35,65.41 20.07,63.12 20.07,61.72 19.43,61.09 17.65,61.09 13.46,56.9 13.46,51.18 10.29,48.01 10.29,47.12 10.92,46.48 10.92,41.78 10.41,41.27 10.41,39.5 11.05,38.86 11.56,38.86 arc-90 12.7,37.85 12.7,32.64 v14.73,30.61
  Bottom 0.305: C4.1 21.97,32.13 19.05,32.13 17.53,30.61 v14.73,30.61
R-STEP1
  Bottom 0.305: R6.2 C4.2
R-STEP2
  Bottom 0.305: VR1.2 12.7,34.65 12.7,33.91 13.34,33.27 15.62,33.27 16.51,34.16 R6.1
R-STEP3  (via drill 0.76 pad 1.27)
  Top 0.305: v45.97,39.24 45.97,39.5 48.26,41.78 49.15,41.78 51.82,44.45 60.71,44.45 61.72,43.43 65.15,43.43 66.42,44.7 67.06,44.7 69.22,46.86 70.87,46.86 71.13,46.6 U4.8
  Bottom 0.305: VR1.4 11.78,31.78 14.22,29.34 23.37,29.34 25.15,31.11 25.15,33.66 30.35,38.86 45.59,38.86 v45.97,39.24
RIGHT  (via drill 0.76 pad 1.27)
  Top 0.305: C9.1 70.1,59.82 68.07,57.78 68.07,53.98 69.22,52.83 73.79,52.83 v75.95,50.67 | U4.12 71.93,33.86 73.41,32.38 74.55,32.38 75.44,33.27 v76.96,33.27
  Bottom 0.305: U$3.3 76.2,1.14 78.61,3.56 78.61,6.22 76.96,7.87 75.31,7.87 75.31,11.91 73.28,13.94 73.28,16.56 76.15,19.43 78.49,19.43 78.49,33.27 v76.96,33.27 76.33,33.91 76.33,42.42 75.18,43.56 75.18,49.91 v75.95,50.67
  pour Bottom (no thermals): 75.69,1.78 76.2,1.78 arc-90 76.71,1.27 76.71,0.76 arc-90 76.2,0.25 75.69,0.25 arc-90 75.18,0.76 75.18,1.27 arc-90
RST  (via drill 0.76 pad 1.27)
  Top 0.305: v42.55,51.44 41.78,50.67 33.78,50.67 31.24,53.34 28.07,53.34 27.12,54.29 U1.71 21.46,54.29 21.46,53.59 19.81,51.94 17.02,51.94 v17.02,52.32 | v57.91,50.29 57.91,54.74 v57.4,55.24
  Bottom 0.305: C10.2 8.26,43.94 8.26,45.85 8.64,46.23 12.57,46.23 13.46,47.12 13.46,50.04 15.75,52.32 v17.02,52.32 | 62.36,69.47 64.77,71.88 64.77,75.67 | R7.1 62.23,69.34 62.36,69.47 | 62.36,69.47 62.36,59.56 63.37,58.55 63.37,54.74 57.4,54.74 | 57.4,54.74 51.56,54.74 48.26,51.44 v42.55,51.44 | v57.91,50.29 58.29,49.91 58.29,37.08 56.13,34.92 56.13,32.89 58.42,30.61 58.42,15.62 55.88,15.62 52.45,19.05 52.45,19.43 51.56,20.32 50.8,20.32 49.91,19.43 49.91,18.67 50.8,17.78 51.69,17.78 55.24,14.22 57.66,14.22 60.75,11.13 60.75,10.5 | v57.4,55.24 57.4,54.74
  pour Bottom (no thermals): 71.63,75.69 64.77,75.69 64.77,73.41 65.53,74.17 71.63,74.17
  pour Top (no thermals): 66.04,75.69 66.04,74.17 71.63,74.17 71.63,75.69
VCC  (via drill 0.64 pad 1.02, 0.76 pad 1.27)
  Top 0.305: U1.58 31.16,65.32 v32.26,66.42
  Top 0.508: 50.29,41.53 U3.28 | U2.28 62.36,66.17 61.72,66.8 v61.09,66.8 | U2.26 62.23,63.63 61.47,64.39 v61.09,64.39
  Top 0.635: 50.8,42.04 50.29,41.53
  Top 0.762: C14.2 57.28,43.18 55.75,41.66 54.1,41.66 53.72,42.04 50.8,42.04
  Bottom 0.305: v32.26,66.42 35.56,66.42
  Bottom 0.762: P3.11 35.56,66.42 35.56,67.69
  Bottom 1.524: U$7.1 75.11,21.34 72.44,18.67 67.18,18.67
  other vias: 60.2,56.01 61.21,56.01 59.56,50.29 60.83,50.29
  pour Bottom (no thermals): 21.34,0.51 21.34,3.3 14.73,3.3 14.73,11.56 17.14,13.97 17.14,23.5 11.56,23.5 10.29,24.77 0.64,24.77 0.64,26.16 7.49,26.16 7.49,40.01 5.08,40.01 3.17,41.91 3.17,47.24 4.45,47.24 5.33,48.13 5.33,49.78 4.45,50.67 3.3,50.67 3.3,58.04 5.46,60.2 5.46,61.47 5.21,61.72 5.21,63.75 6.22,64.77 6.22,67.18 5.08,68.33 5.08,73.53 0.64,73.53 0.64,77.72 60.71,77.72 60.71,70.87 60.07,70.87 arc180 60.07,67.82 61.59,67.82 61.59,59.56 62.61,58.42 62.61,55.5 59.56,55.5 59.56,56.01 60.58,56.9 60.58,58.67 59.18,60.07 57.78,60.07 57.78,64.52 55.75,64.52 55.75,74.8 50.16,74.8 arc35 49.02,75.18 40.01,75.18 arc90 38.61,73.66 38.61,72.01 36.32,72.01 arc150 35.81,69.11 35.81,65.53 35.18,65.53 34.67,66.04 32.77,66.04 32,66.8 33.53,68.33 33.53,70.1 30.73,72.9 30.73,74.55 30.35,74.93 23.75,74.93 23.11,74.3 23.11,72.9 20.07,72.9 20.07,71.63 8.89,71.63 8.89,58.67 5.08,58.67 4.32,57.91 4.32,51.94 5.21,51.05 7.37,51.05 7.37,45.34 6.6,45.34 arc180 6.6,42.55 9.91,42.55 9.91,41.15 11.94,41.15 11.94,39.62 9.91,39.62 9.91,29.34 10.92,28.32 11.94,28.32 11.94,26.42 12.32,26.04 19.56,26.04 19.56,13.21 17.14,10.79 17.14,7.11 arc-90 17.78,6.6 17.78,4.57 62.36,4.57 65.02,7.24 65.02,24.38 60.71,28.7 60.71,35.05 59.05,36.7 59.05,50.8 61.34,50.8 61.34,44.58 62.99,42.93 62.99,29.59 67.56,25.02 67.56,18.03 66.42,16.89 66.42,14.48 66.29,14.35 66.29,3.17 59.94,3.17 59.94,0.51
  pour Top: 62.23,49.66 59.18,49.66 59.18,50.8 58.55,51.56 58.55,54.99 60.2,56.64 61.21,56.64 62.23,55.63
(copper drawn outside any net)
  shapes: Bottom circle x6, Top area x3, Top circle x4

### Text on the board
tSilk: SW1 | 3 | 4 | DA1 | DA2 | DA3 | DA4 | 4-DA216 | C12 | C6 | /10V | 0.01µ | 10µ/16V | 180K | 100µ | C13 | C1 | 220 | MAIN SW | 0.01µ | R7 | 180K | U2 | 2 | 1 | R4 | 220 | C18 | C19 | C16 | DMG CPU | C20 | C17 | 2 | 6 | 64K | 1 | DC | 3-220 | C9 | P2 | R1 | D1 | 220 | 5 | R2 | 0.047µ | 220 | 3 | R3 | 220 | S-RAM | RB100A | 4 | 1 | U2 | 27P | U1 | 0.047µ | 3 | 254 | C21 | 0.047µ | DMG CPU | C2 | 2 | C11 | ISS | U1 | 64K S-RAM | C8 | C7 | 0.01µ | 0.01µ | 1M | C14 | 100µ | /10V | D2 | X1 | AMP | C10 | 0.1µ | 4.194304MHz | U3 | 114 | VR1 | 1M | DMG | R8 | 27 | C3 | DMG AMP | 1µ/50V | U3 | P | VR1 / 10K×2 | C22 | U4 | R6 | 64K | 510 | 510 | 64K | S-RAM | /16V | C4 | S-RAM | 510 | 510 | C5 | 10µ | R5 | 1µ/50V | G | C15 / 10Kx2 | 0.01µ | N | P1 | B | DMG-CPU-06
Notes: 0 | 1 | 2 | 3 | 4 | 5 | 6 | 7 | 8 | 9 | I | I | H | H | G | G | F | F | E | E | D | D | C | C | B | B | A | A | 0.5 in | X | X | 1 cm | 0 | 1 | 2 | 3 | 4 | 5 | 6 | 7 | 8 | 9 | Nintindo®, Game Boy®, and the information depicted here are registered trademarks or intellectual property of Nintindo Co., Ltd. / If you are not the copyright holder, your usage of this work is licensed under a Creative Commons Attribution-NonCommercial-NoDerivatives 4.0 (or later) International License.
